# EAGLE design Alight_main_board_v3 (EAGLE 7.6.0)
CNAME: Alarm Light Main board / Juraj Repcik; CREVISION: 03
Assembly variants: ESP8266 CH340 default

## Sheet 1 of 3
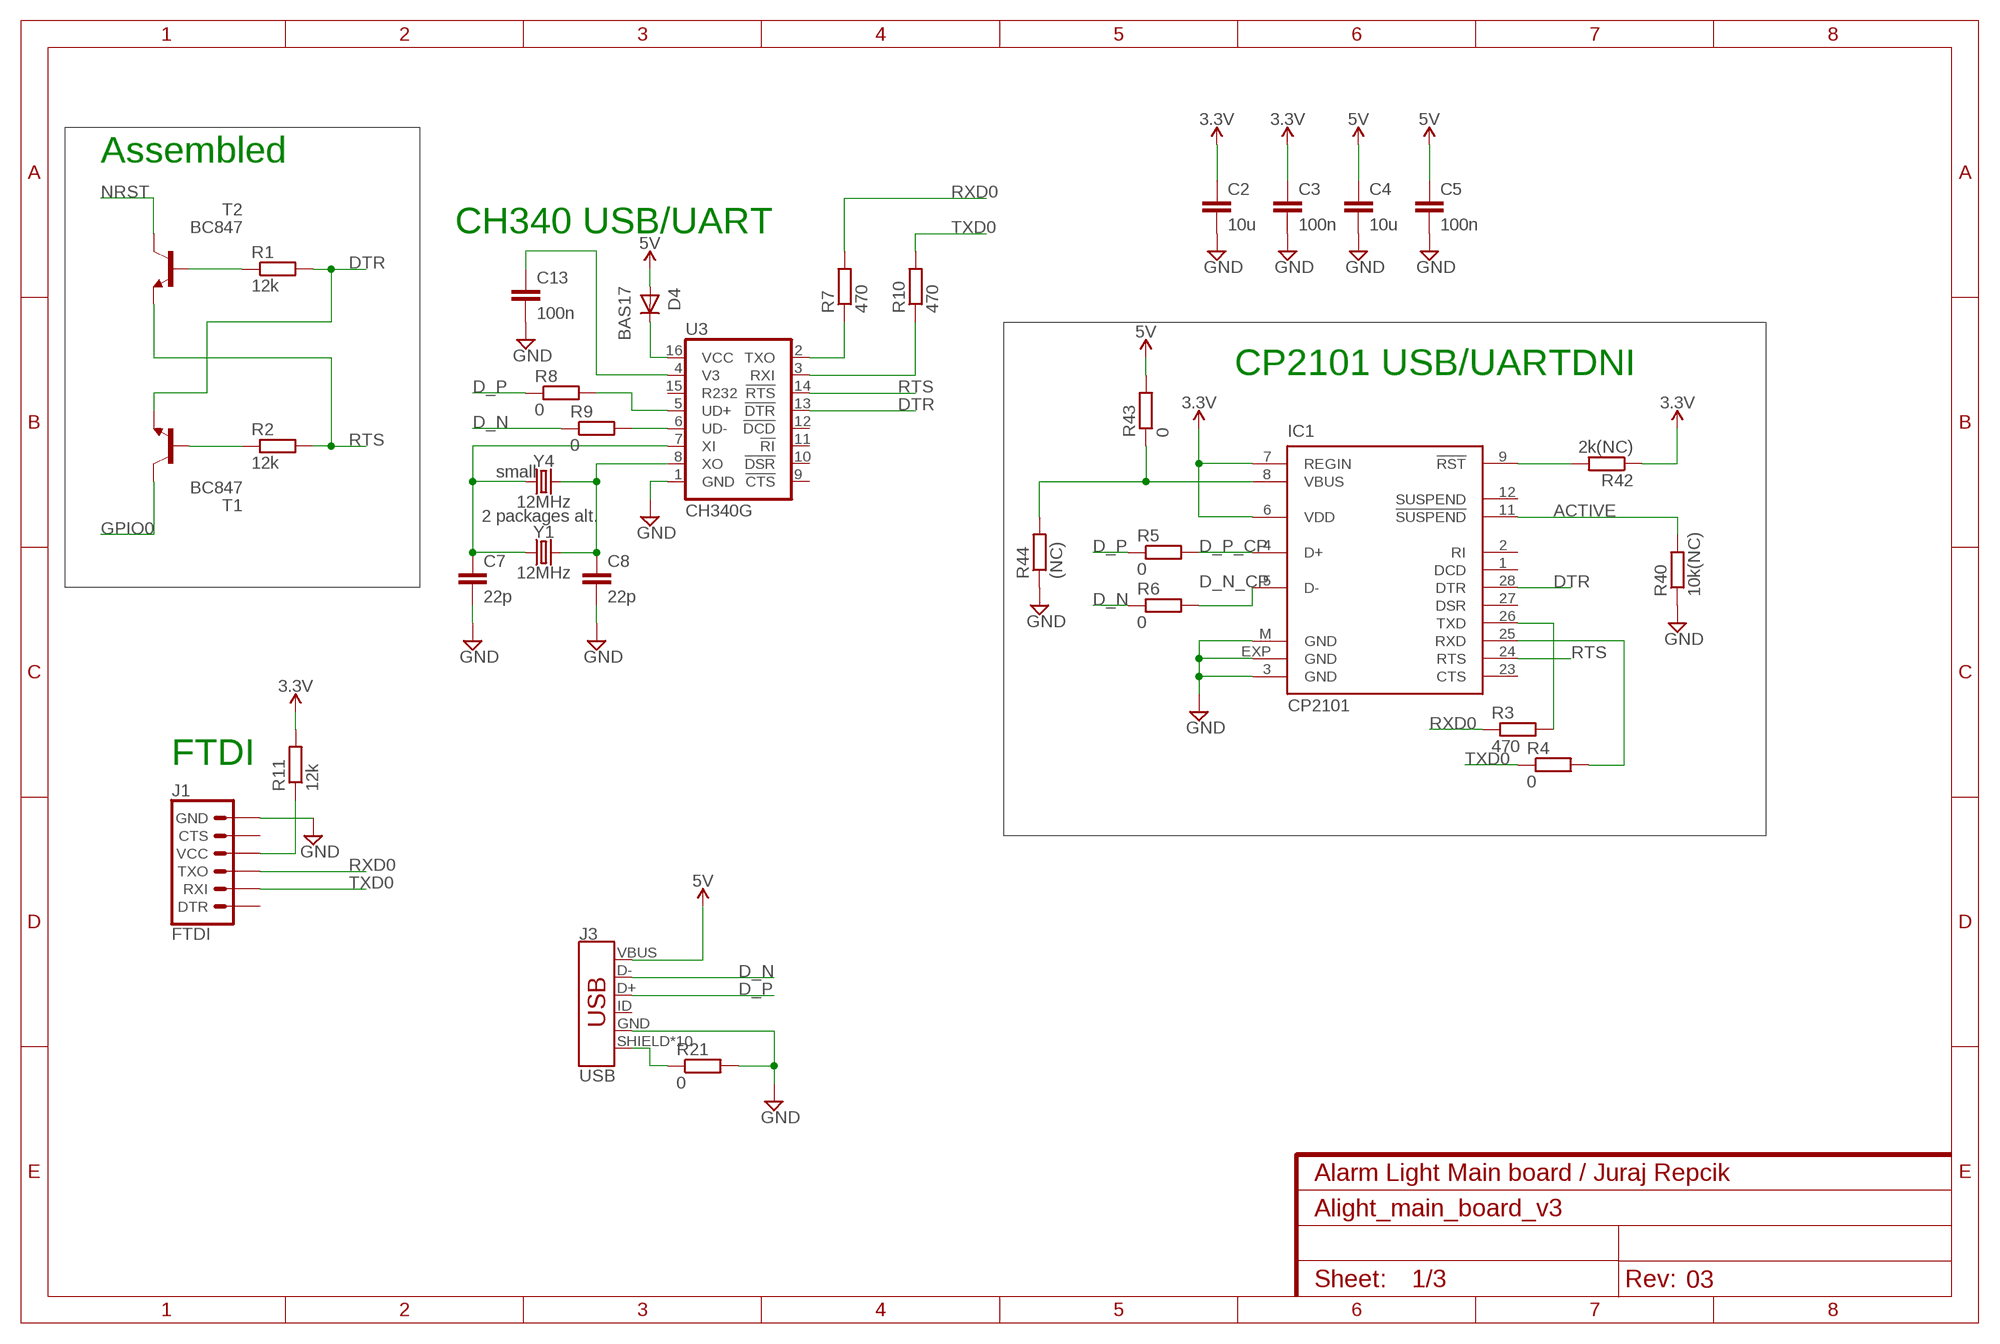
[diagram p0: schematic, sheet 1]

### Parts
C2  10u  C-EUC0603K  [C0603K]
C3  100n  C-EUC0603K  [C0603K]
C4  10u  C-EUC0603K  [C0603K]
C5  100n  C-EUC0603K  [C0603K]
C7  22p  C-EUC0402  [C0402]
C8  22p  C-EUC0402  [C0402]
C13  100n  C-EUC0603K  [C0603K]
D4  BAS17  [SOT23]
IC1  CP2101  CP210X_USB_UART  [MLP28]  (not fitted in variant ESP8266 CH340 default)
J1  FTDI  6_PIN_SERIAL_TARGETLONGPADS  [1X06_LONGPADS]
J3  USB  USB_MICRO-B_HALF_PTH_MILL  [USB-MICROB-PTH-MILL]
R1  12k  R-EU_R0603  [R0603]
R2  12k  R-EU_R0603  [R0603]
R3  470  R-EU_R0603  [R0603]  (not fitted in variant ESP8266 CH340 default)
R4  0  R-EU_R0603  [R0603]  (not fitted in variant ESP8266 CH340 default)
R5  0  R-EU_R0603  [R0603]  (not fitted in variant ESP8266 CH340 default)
R6  0  R-EU_R0603  [R0603]  (not fitted in variant ESP8266 CH340 default)
R7  470  R-EU_R0603  [R0603]
R8  0  R-EU_R0603  [R0603]
R9  0  R-EU_R0603  [R0603]
R10  470  R-EU_R0603  [R0603]
R11  12k  R-EU_R0603  [R0603]
R21  0  R-EU_R0603  [R0603]
R40  10k(NC)  R-EU_R0603  [R0603]  (not fitted in variant ESP8266 CH340 default)
R42  2k(NC)  R-EU_R0603  [R0603]  (not fitted in variant ESP8266 CH340 default)
R43  0  R-EU_R0603  [R0603]  (not fitted in variant ESP8266 CH340 default)
R44  (NC)  R-EU_R0603  [R0603]  (not fitted in variant ESP8266 CH340 default)
T1  BC847  [SOT23]
T2  BC847  [SOT23]
U3  CH340G  CH340GSMD  [SO016]
Y1  12MHz  CRYSTALSMD-HC49UP  [HC49UP]
Y4  12MHz  CRYSTAL-32.768KHZSMD-3.2X1.5  [CRYSTAL-SMD-3.2X1.5MM]  (not fitted in variant ESP8266 CH340 default)

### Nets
3.3V: C2.1 C3.1 IC1.6(VDD) IC1.7(REGIN) R11.2 R42.1 ; also sheet 2,3
5V: C4.1 C5.1 D4.1(A) J3.VBUS R43.2 ; also sheet 2,3
ACTIVE: IC1.11(!SUSPEND) R40.2
D_N: J3.D- R6.1 R9.1
D_N_CP: IC1.5(D-) R6.2
D_P: J3.D+ R5.1 R8.1
D_P_CP: IC1.4(D+) R5.2
DTR: IC1.28(DTR) R1.2 T1.2(E) U3.13(!DTR)
GND: C2.2 C3.2 C4.2 C5.2 C7.2 C8.2 C13.2 IC1.3(GND) IC1.EXP(GND) IC1.M(GND) J1.6(GND) J3.GND R21.2 R40.1 R44.1 U3.1(GND) ; also sheet 2,3
GPIO0: T1.3(C) ; also sheet 2
N$1: R1.1 T2.1(B)
N$2: R2.1 T1.1(B)
N$4: R7.1 U3.2(TXO)
N$5: R10.1 U3.3(RXI)
N$6: R8.2 U3.5(UD+)
N$7: R9.2 U3.6(UD-)
N$8: C7.1 U3.7(XI) Y1.1 Y4.P$1
N$9: C13.1 U3.4(V3)
N$10: C8.1 U3.8(XO) Y1.2 Y4.P$2
N$11: J1.4(VCC) R11.1
N$15: D4.3(K) U3.16(VCC)
N$38: IC1.9(!RST) R42.2
N$39: IC1.8(VBUS) R43.1 R44.2
NRST: T2.3(C) ; also sheet 2,3
RTS: IC1.24(RTS) R2.2 T2.2(E) U3.14(!RTS)
RXD0: J1.3(TXO) R3.1 R7.2 ; also sheet 2,3
RXD0_CP2101IN: IC1.26(TXD) R3.2
SHIELD: J3.SHIELD J3.SHIELD2(SHIELD) J3.SHIELD3(SHIELD) J3.SHIELD4(SHIELD) J3.SHIELD5(SHIELD) J3.SHIELD6(SHIELD) J3.SHIELD7(SHIELD) J3.SHIELD8(SHIELD) J3.SHIELD9(SHIELD) J3.SHIELD10(SHIELD) R21.1
TXD0: J1.2(RXI) R4.1 R10.2 ; also sheet 2,3
TXD0_CP2101: IC1.25(RXD) R4.2
Unconnected: IC1.1(DCD) IC1.2(RI) IC1.12(SUSPEND) IC1.23(CTS) IC1.27(DSR) J1.1(DTR) J1.5(CTS) J3.ID U3.9(!CTS) U3.10(!DSR) U3.11(!RI) U3.12(!DCD) U3.15(R232)

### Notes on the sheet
- Assembled
- CH340 USB/UART
- CP2101 USB/UART | DNI
- small
- 2 packages alt.
- FTDI

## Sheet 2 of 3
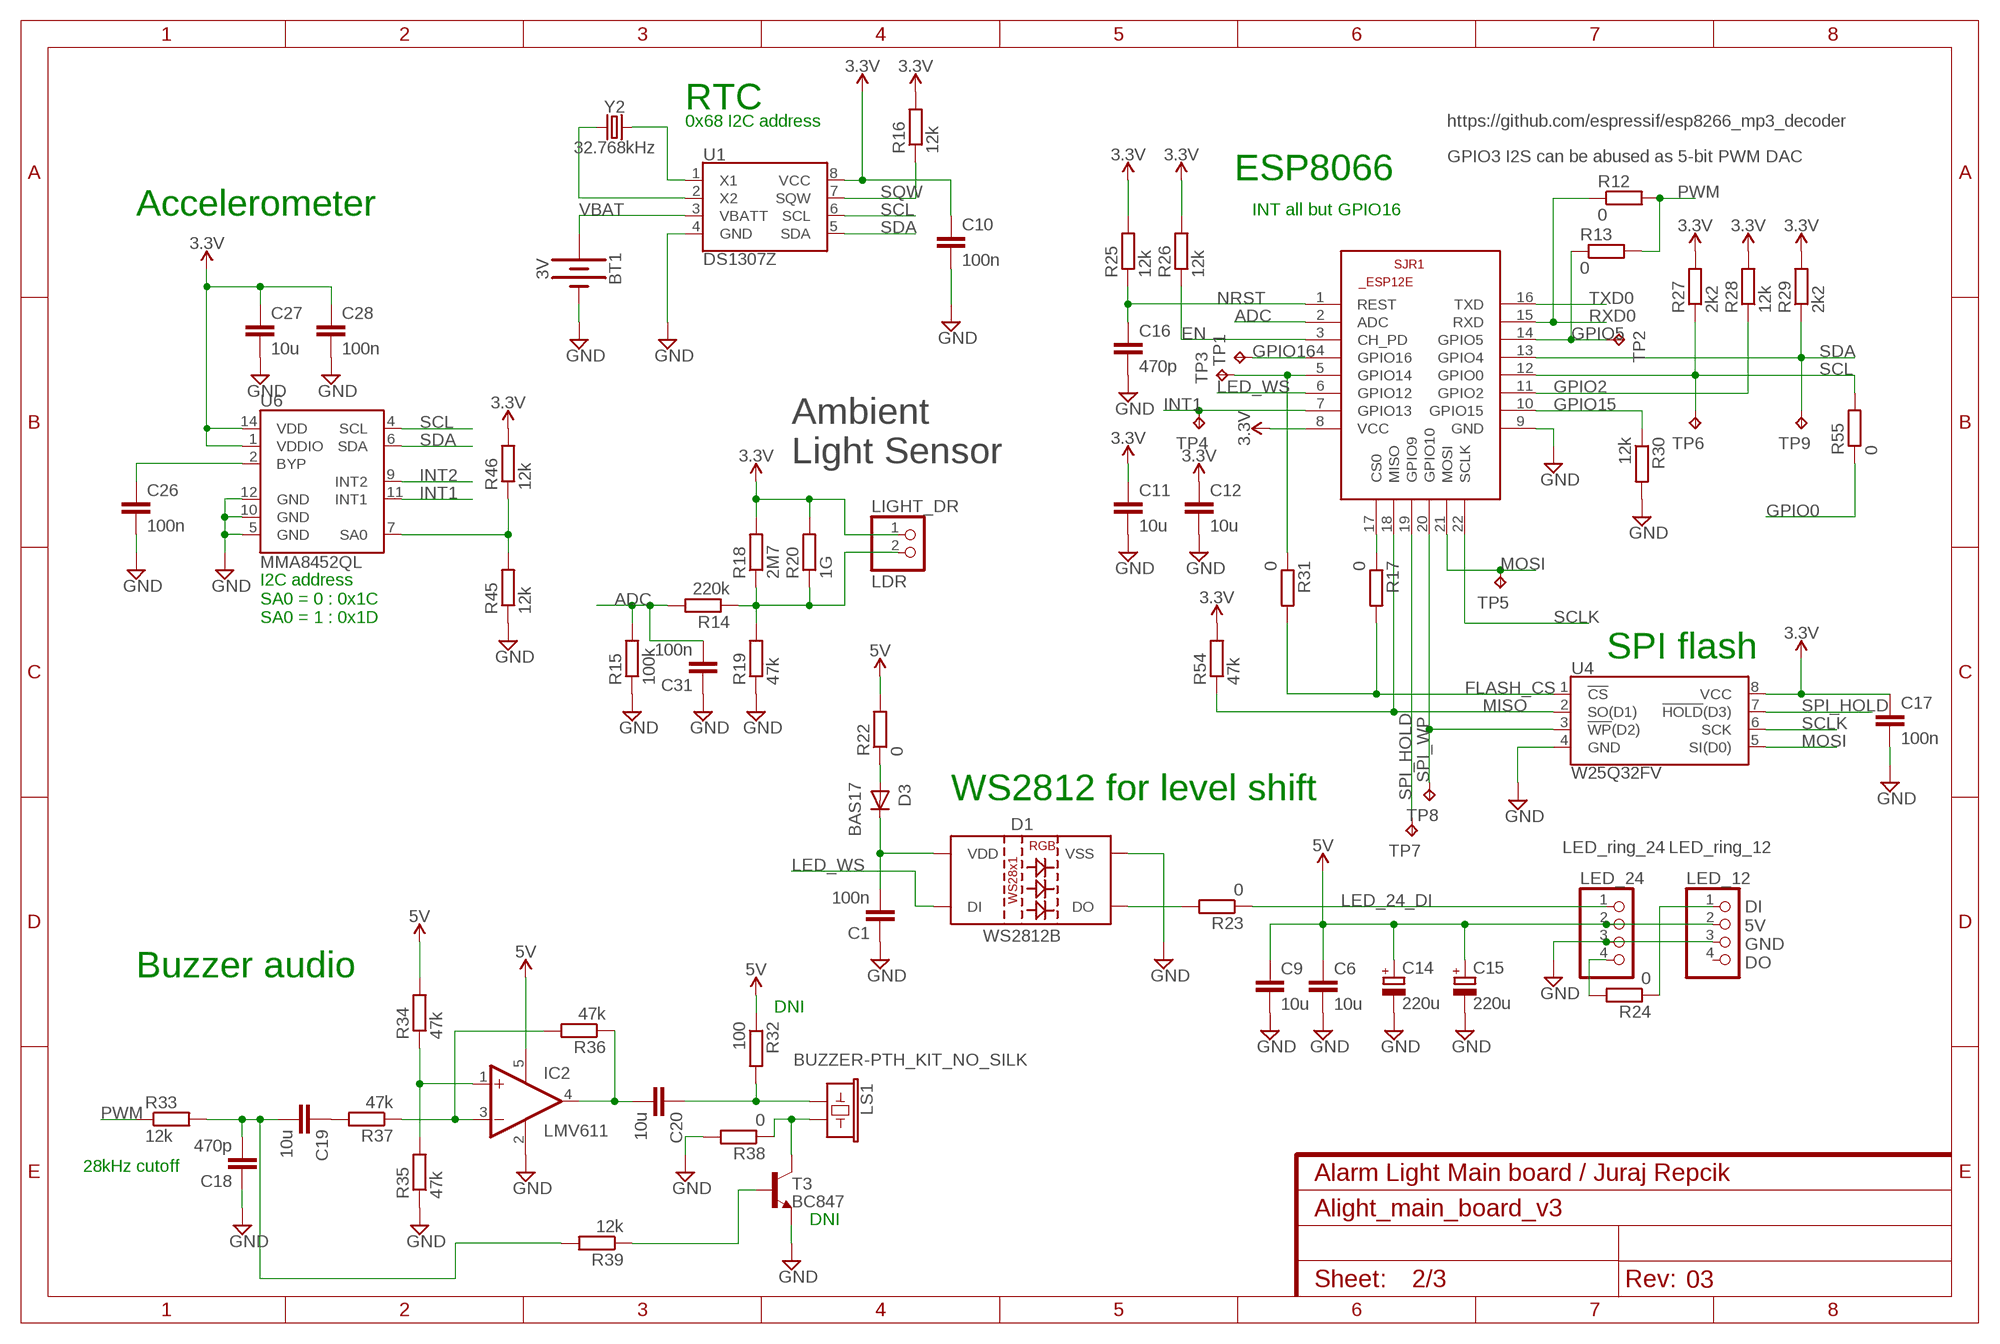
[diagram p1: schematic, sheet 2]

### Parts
BT1  3V  BATTERY-20MM_PTH_KIT  [BATTCOM_20MM_PTH_KIT]
C1  100n  C-EUC0603K  [C0603K]
C6  10u  C-EUC0603K  [C0603K]
C9  10u  C-EUC0603K  [C0603K]
C10  100n  C-EUC0603K  [C0603K]
C11  10u  C-EUC0603K  [C0603K]
C12  10u  C-EUC0603K  [C0603K]
C14  220u  CPOL-EU153CLV-0605  [153CLV-0605]
C15  220u  CPOL-EU153CLV-0605  [153CLV-0605]
C16  470p  C-EUC0603K  [C0603K]
C17  100n  C-EUC0603K  [C0603K]  (not fitted in variant ESP8266 CH340 default)
C18  470p  C-EUC0603K  [C0603K]
C19  10u  C-EUC0603K  [C0603K]
C20  10u  C-EUC0603K  [C0603K]
C26  100n  C-EUC0603K  [C0603K]
C27  10u  C-EUC0603K  [C0603K]
C28  100n  C-EUC0603K  [C0603K]
C31  100n  C-EUC0603K  [C0603K]
D1  WS2812B  [WS2812B]
D3  BAS17  [SOT23]
IC2  LMV611  OPA333DCK  [SC70-5L]
LED_12  LED_ring_12  PINHD-1X4  [1X04]
LED_24  LED_ring_24  PINHD-1X4  [1X04]
LIGHT_DR  LDR  PINHD-1X2  [1X02]
LS1  BUZZER-PTH_KIT_NO_SILK  [BUZZER-12MM-NS-KIT]
R12  0  R-EU_R0603  [R0603]  (not fitted in variant ESP8266 CH340 default)
R13  0  R-EU_R0603  [R0603]
R14  220k  R-EU_R0603  [R0603]
R15  100k  R-EU_R0603  [R0603]
R16  12k  R-EU_R0603  [R0603]
R17  0  R-EU_R0603  [R0603]  (not fitted in variant ESP8266 CH340 default)
R18  2M7  R-EU_R0603  [R0603]
R19  47k  R-EU_R0603  [R0603]
R20  1G  R-EU_R0603  [R0603]  (not fitted in variant ESP8266 CH340 default)
R22  0  R-EU_R0603  [R0603]
R23  0  R-EU_R0603  [R0603]
R24  0  R-EU_R0603  [R0603]
R25  12k  R-EU_R0603  [R0603]
R26  12k  R-EU_R0603  [R0603]
R27  2k2  R-EU_R0603  [R0603]
R28  12k  R-EU_R0603  [R0603]
R29  2k2  R-EU_R0603  [R0603]
R30  12k  R-EU_R0603  [R0603]
R31  0  R-EU_R0603  [R0603]  (not fitted in variant ESP8266 CH340 default)
R32  100  R-EU_R0603  [R0603]  (not fitted in variant ESP8266 CH340 default)
R33  12k  R-EU_R0603  [R0603]
R34  47k  R-EU_R0603  [R0603]
R35  47k  R-EU_R0603  [R0603]
R36  47k  R-EU_R0603  [R0603]
R37  47k  R-EU_R0603  [R0603]
R38  0  R-EU_R0603  [R0603]
R39  12k  R-EU_R0603  [R0603]  (not fitted in variant ESP8266 CH340 default)
R45  12k  R-EU_R0603  [R0603]  (not fitted in variant ESP8266 CH340 default)
R46  12k  R-EU_R0603  [R0603]
R54  47k  R-EU_R0603  [R0603]  (not fitted in variant ESP8266 CH340 default)
R55  0  R-EU_R0603  [R0603]
SJR1  ESP12E/F  ESP8266-12EESP12E  [ESP8266-ESP12E]
T3  BC847  [SOT23]  (not fitted in variant ESP8266 CH340 default)
TP1  TPTP10R  [TP10R]
TP2  TPTP10R  [TP10R]
TP3  TPTP10R  [TP10R]
TP4  TPTP10R  [TP10R]
TP5  TPTP10R  [TP10R]
TP6  TPTP10R  [TP10R]
TP7  TPTP10R  [TP10R]
TP8  TPTP10R  [TP10R]
TP9  TPTP10R  [TP10R]
U1  DS1307Z  [SO08-0.15]
U4  W25Q32FV  W25Q32FVSS  [SOIC-8]  (not fitted in variant ESP8266 CH340 default)
U6  MMA8452QL  [QFN-16_0.5MM-EXTRA]
Y2  32.768kHz  CRYSTAL-32.768KHZSMD-3.2X1.5  [CRYSTAL-SMD-3.2X1.5MM]

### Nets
3.3V: C10.1 C11.1 C12.1 C17.1 C27.1 C28.1 LIGHT_DR.1 R16.2 R18.2 R20.2 R25.2 R26.2 R27.2 R28.2 R29.2 R46.2 R54.2 SJR1.8(VCC) U1.8(VCC) U4.8(VCC) U6.1(VDDIO) U6.14(VDD) ; also sheet 1,3
5V: C6.1 C9.1 C14.+ C15.+ IC2.5(V+) LED_12.2 LED_24.2 R22.2 R32.1 R34.2 ; also sheet 1,3
ADC: C31.2 R14.2 R15.2 SJR1.2(ADC) ; also sheet 3
EN: R26.1 SJR1.3(CH_PD)
FLASH_CS: R17.2 R31.2 U4.1(!CS!) ; also sheet 3
GND: BT1.2(-) C1.1 C6.2 C9.2 C10.2 C11.2 C12.2 C14.- C15.- C16.2 C17.2 C18.1 C26.2 C27.2 C28.2 C31.1 D1.3(VSS) IC2.2(V-) LED_12.3 LED_24.3 R15.1 R19.1 R30.2 R35.1 R38.2 R45.1 SJR1.9(GND) T3.2(E) U1.4(GND) U4.4(GND) U6.5(GND) U6.10(GND) U6.12(GND) ; also sheet 1,3
GPIO0: R55.1 ; also sheet 1
GPIO2: R28.1 SJR1.11(GPIO2) ; also sheet 3
GPIO5: R13.1 SJR1.14(GPIO5) TP2.TP
GPIO15: R30.1 SJR1.10(GPIO15)
GPIO16: SJR1.4(GPIO16) TP1.TP
INT1: SJR1.7(GPIO13) TP4.TP U6.11(INT1) ; also sheet 3
INT2: U6.9(INT2) ; also sheet 3
LED_12DI: LED_12.1 R24.1
LED_24_DI: LED_24.1 R23.1
LED_24_DO: LED_24.4 R24.2
LED_WS: D1.4(DI) SJR1.6(GPIO12) ; also sheet 3
MISO: R54.1 SJR1.18(MISO) U4.2(SO(D1))
MOSI: SJR1.21(MOSI) TP5.TP U4.5(SI(D0))
N$3: C1.2 D1.1(VDD) D3.3(K)
N$14: LIGHT_DR.2 R14.1 R18.1 R19.2 R20.1
N$16: D3.1(A) R22.1
N$18: D1.2(DO) R23.2
N$19: C26.1 U6.2(BYP)
N$21: R31.1 SJR1.5(GPIO14) TP3.TP
N$22: R17.1 SJR1.17(CS0)
N$25: LS1.- R38.1 T3.3(C)
N$26: R39.1 T3.1(B)
N$28: IC2.1(+IN) R34.1 R35.2
N$30: U1.1(X1) Y2.P$2
N$31: U1.2(X2) Y2.P$1
N$32: IC2.3(-IN) R36.2 R37.1
N$33: C20.1 LS1.+ R32.2
N$34: C19.1 R37.2
N$35: C20.2 IC2.4(OUT) R36.1
N$36: C18.2 C19.2 R33.2 R39.2
N$40: R45.2 R46.1 U6.7(SA0)
NRST: C16.1 R25.1 SJR1.1(REST) ; also sheet 1,3
PWM: R12.2 R13.2 R33.1 ; also sheet 3
RXD0: R12.1 SJR1.15(RXD) ; also sheet 1,3
SCL: R27.1 R55.2 SJR1.12(GPIO0) TP6.TP U1.6(SCL) U6.4(SCL) ; also sheet 3
SCLK: SJR1.22(SCLK) U4.6(SCK)
SDA: R29.1 SJR1.13(GPIO4) TP9.TP U1.5(SDA) U6.6(SDA) ; also sheet 3
SPI_HOLD: SJR1.19(GPIO9) TP7.TP U4.7(!HOLD!(D3))
SPI_WP: SJR1.20(GPIO10) TP8.TP U4.3(!WP!(D2))
SQW: R16.1 U1.7(SQW)
TXD0: SJR1.16(TXD) ; also sheet 1,3
VBAT: BT1.1(+) U1.3(VBATT)
Unconnected: LED_12.4

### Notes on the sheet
- RTC
- 0x68 I2C address | https://github.com/espressif/esp8266_mp3_decoder
- GPIO3 I2S can be abused as 5-bit PWM DAC
- ESP8066
- Accelerometer | INT all but GPIO16
- Ambient
  Light Sensor
- I2C address
  SA0 = 0 : 0x1C
  SA0 = 1 : 0x1D
- SPI flash
- WS2812 for level shift
- DI
  5V
  GND
  DO
- Buzzer audio
- DNI
- 28kHz cutoff
- DNI

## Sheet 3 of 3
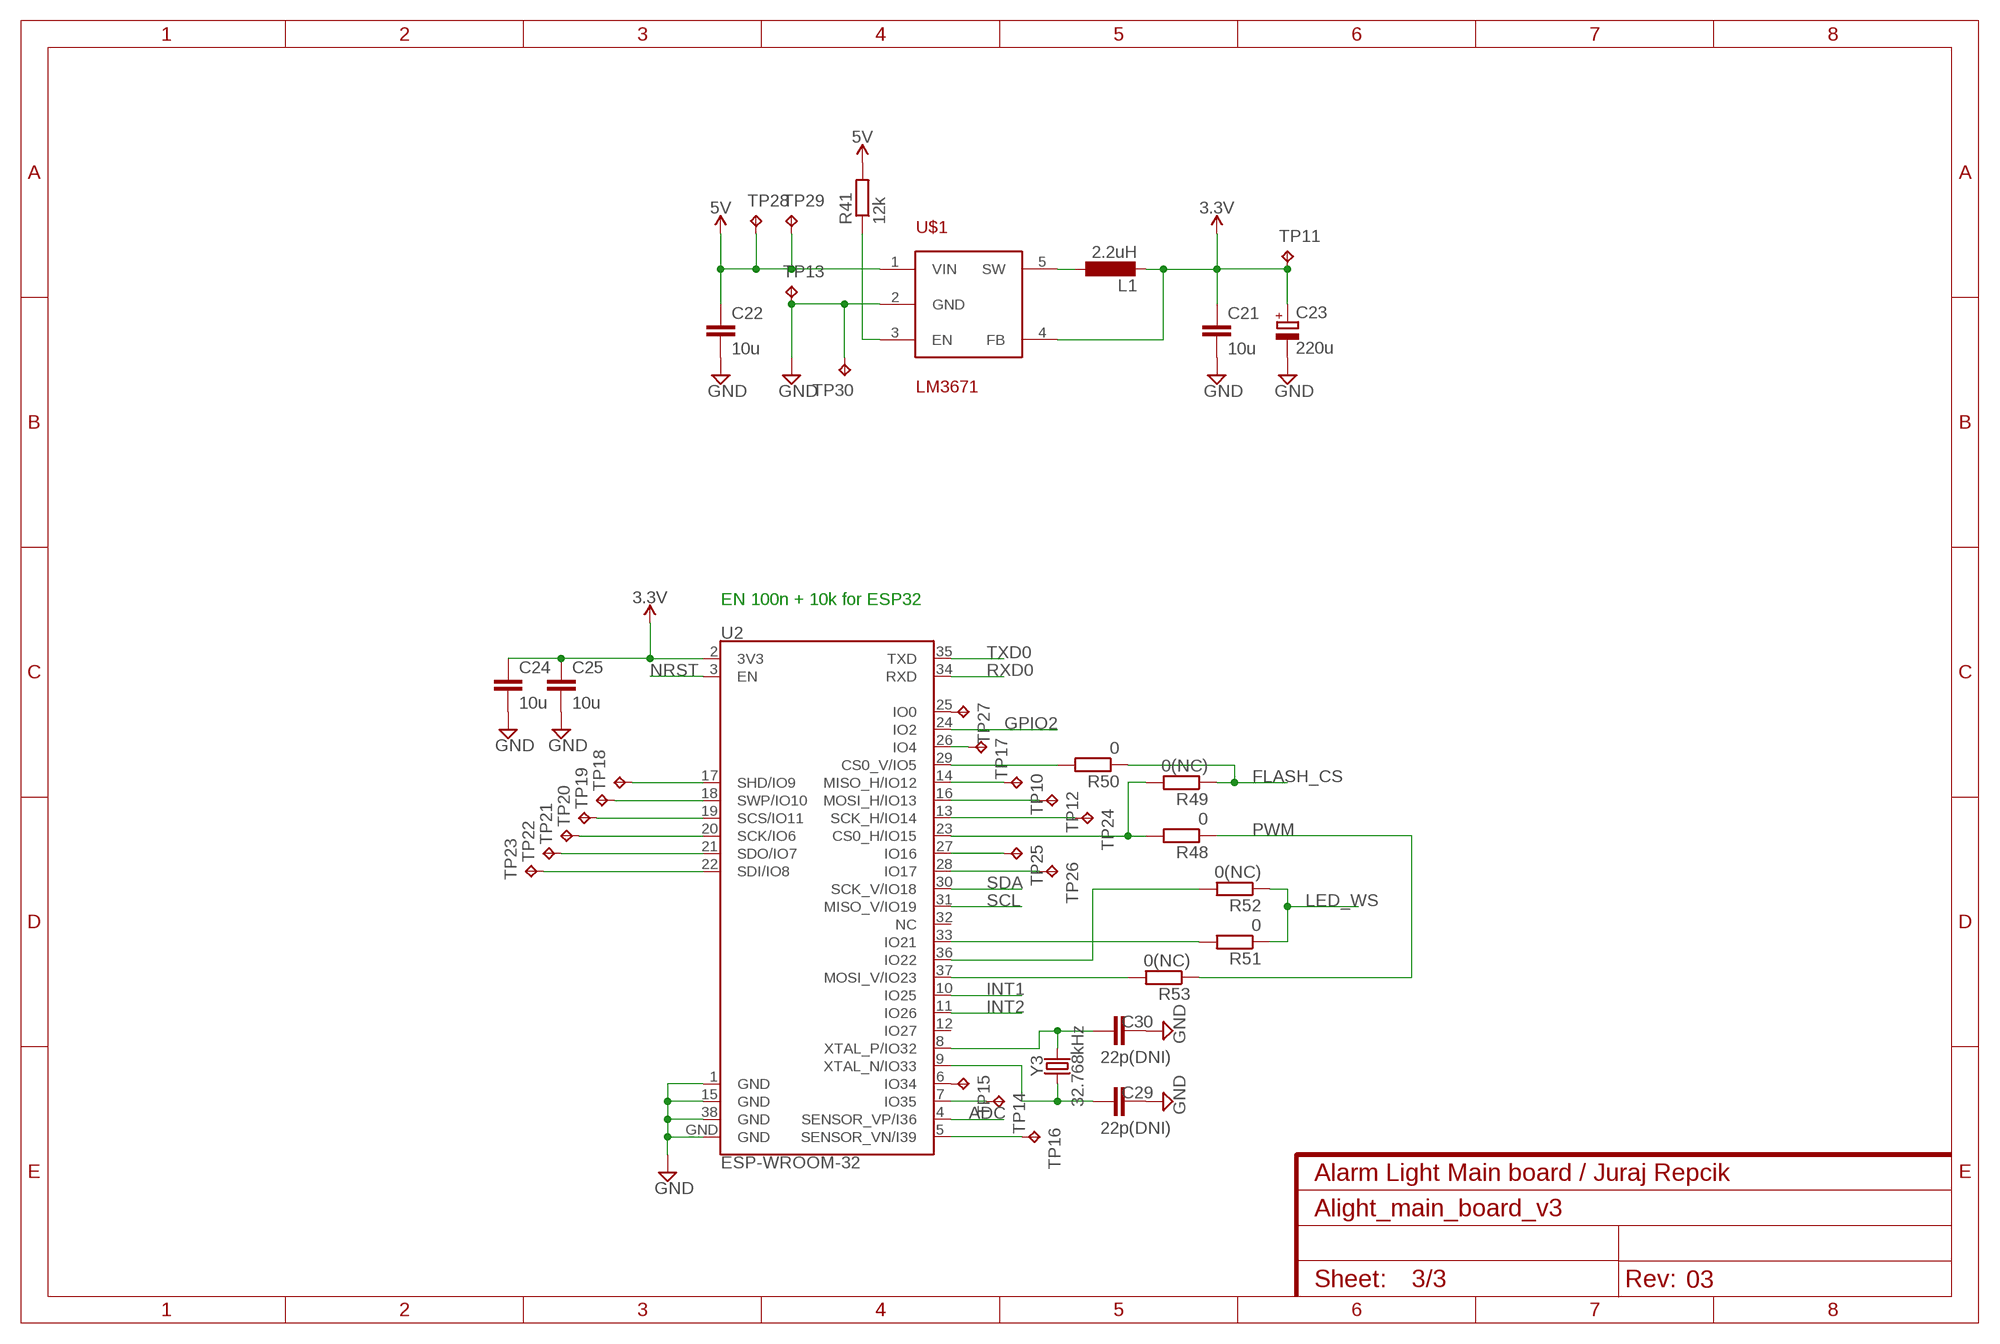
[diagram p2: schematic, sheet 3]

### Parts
C21  10u  C-EUC0603K  [C0603K]
C22  10u  C-EUC0603K  [C0603K]
C23  220u  CPOL-EU153CLV-0605  [153CLV-0605]
C24  10u  C-EUC0603K  [C0603K]  (not fitted in variant ESP8266 CH340 default)
C25  10u  C-EUC0603K  [C0603K]  (not fitted in variant ESP8266 CH340 default)
C29  22p(DNI)  C-EUC0402  [C0402]  (not fitted in variant ESP8266 CH340 default)
C30  22p(DNI)  C-EUC0402  [C0402]  (not fitted in variant ESP8266 CH340 default)
L1  2.2uH  L-EUL3225M  [L3225M]
R41  12k  R-EU_R0603  [R0603]
R48  0  R-EU_R0603  [R0603]  (not fitted in variant ESP8266 CH340 default)
R49  0(NC)  R-EU_R0603  [R0603]  (not fitted in variant ESP8266 CH340 default)
R50  0  R-EU_R0603  [R0603]  (not fitted in variant ESP8266 CH340 default)
R51  0  R-EU_R0603  [R0603]  (not fitted in variant ESP8266 CH340 default)
R52  0(NC)  R-EU_R0603  [R0603]  (not fitted in variant ESP8266 CH340 default)
R53  0(NC)  R-EU_R0603  [R0603]  (not fitted in variant ESP8266 CH340 default)
TP10  TPTP10R  [TP10R]
TP11  TPTP10R  [TP10R]
TP12  TPTP10R  [TP10R]
TP13  TPTP10R  [TP10R]
TP14  TPTP10R  [TP10R]
TP15  TPTP10R  [TP10R]
TP16  TPTP10R  [TP10R]
TP17  TPTP10R  [TP10R]
TP18  TPTP10R  [TP10R]
TP19  TPTP10R  [TP10R]
TP20  TPTP10R  [TP10R]
TP21  TPTP10R  [TP10R]
TP22  TPTP10R  [TP10R]
TP23  TPTP10R  [TP10R]
TP24  TPTP10R  [TP10R]
TP25  TPTP10R  [TP10R]
TP26  TPTP10R  [TP10R]
TP27  TPTP10R  [TP10R]
TP28  TPTP10R  [TP10R]
TP29  TPTP10R  [TP10R]
TP30  TPTP10R  [TP10R]
U2  ESP-WROOM-32  [ESP-WROOM-32]  (not fitted in variant ESP8266 CH340 default)
U$1  LM3671  [SOT23-5]
Y3  32.768kHz  CRYSTAL-32.768KHZSMD-3.2X1.5  [CRYSTAL-SMD-3.2X1.5MM]  (not fitted in variant ESP8266 CH340 default)

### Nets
3.3V: C21.1 C23.+ C24.1 C25.1 L1.2 TP11.TP U2.2(3V3) U$1.4(FB) ; also sheet 1,2
5V: C22.1 R41.2 TP28.TP TP29.TP U$1.1(VIN) ; also sheet 1,2
ADC: U2.4(SENSOR_VP/I36) ; also sheet 2
FLASH_CS: R49.1 R50.1 ; also sheet 2
GND: C21.2 C22.2 C23.- C24.2 C25.2 C29.2 C30.2 TP13.TP TP30.TP U2.1(GND) U2.15(GND) U2.38(GND) U2.GND U$1.2(GND) ; also sheet 1,2
GPIO2: U2.24(IO2) ; also sheet 2
INT1: U2.10(IO25) ; also sheet 2
INT2: U2.11(IO26) ; also sheet 2
LED_WS: R51.1 R52.1 ; also sheet 2
N$12: C30.1 U2.8(XTAL_P/IO32) Y3.P$2
N$13: C29.1 U2.9(XTAL_N/IO33) Y3.P$1
N$20: R48.2 R49.2 U2.23(CS0_H/IO15)
N$23: R51.2 U2.33(IO21)
N$24: R52.2 U2.36(IO22)
N$27: R41.1 U$1.3(EN)
N$37: L1.1 U$1.5(SW)
N$41: R50.2 U2.29(CS0_V/IO5)
N$42: R53.2 U2.37(MOSI_V/IO23)
N$43: TP14.TP U2.7(IO35)
N$44: TP15.TP U2.6(IO34)
N$45: TP16.TP U2.5(SENSOR_VN/I39)
N$46: TP17.TP U2.26(IO4)
N$47: TP18.TP U2.17(SHD/IO9)
N$48: TP19.TP U2.18(SWP/IO10)
N$49: TP20.TP U2.19(SCS/IO11)
N$50: TP21.TP U2.20(SCK/IO6)
N$51: TP22.TP U2.21(SDO/IO7)
N$52: TP23.TP U2.22(SDI/IO8)
N$63: TP10.TP U2.14(MISO_H/IO12)
N$64: TP12.TP U2.16(MOSI_H/IO13)
N$65: TP24.TP U2.13(SCK_H/IO14)
N$66: TP25.TP U2.27(IO16)
N$67: TP26.TP U2.28(IO17)
N$68: TP27.TP U2.25(IO0)
NRST: U2.3(EN) ; also sheet 1,2
PWM: R48.1 R53.1 ; also sheet 2
RXD0: U2.34(RXD) ; also sheet 1,2
SCL: U2.31(MISO_V/IO19) ; also sheet 2
SDA: U2.30(SCK_V/IO18) ; also sheet 2
TXD0: U2.35(TXD) ; also sheet 1,2
Unconnected: U2.12(IO27) U2.32(NC)

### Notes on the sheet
- EN 100n + 10k for ESP32

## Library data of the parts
BT1 = SparkFun-Batteries:BATTERY: Battery - Single Cell
C1-C13 C16-C22 C24-C31 = resistor:C-EU: CAPACITOR, European symbol
C14 C15 C23 = resistor:CPOL-EU: POLARIZED CAPACITOR, European symbol
D1 = SparkFun-LED:WS2812B: WS2812B SMD addressable RGB LED 5x5mm SMD LED with built-in controller IC. Color: Red/Green/Blue mC Rating: RGB: 390, 660, 180 mcd Forward Voltage: RGB: 2.0, 3.0, 3.0 V Packages:WS2812B SparkFun Products: Blynk Board - ESP8266; PROD_ID: DIO-12503
D3 D4 = nxp_60:BAS17: Low-voltage stabistor
IC1 = SparkFun-Retired:CP210X_USB_UART: Single-Chip USB to UART Bridge Source: www.silabs.com .. CP2101.pdf / cp2102.pdf. Spark Fun Electronics SKU : COM-00310 RETIRED: IC-00865; PROD_ID: COM-00310
IC2 = linear:OPA333: 1.8V, microPOWER CMOS OPERATIONAL AMPLIFIERS Zerø-Drift Series Source: Texas Instruments (Burr-Brown) .. U11 opa333 Operational Amp.pdf
J1 = SparkFun-Connectors:6_PIN_SERIAL_TARGET: 6-pin header connection for use with the "FTDI BASIC" pinout - TARGET SIDE. Also known as "Arduino Serial Program Header". It is used to mate with our FTDI Basic serial programmers using the Arduino IDE. Note, this device has "TARGET" in the name. It is intended to be used on a design that contains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
J3 = SparkFun-Connectors:USB_MICRO-B: USB Type Micro-B Connector Male/female and PTH/SMT variants SparkFun Products: SparkFun microB USB Breakout SparkFun USB microB Plug Breakout SparkFun ESP8266 Thing; PROD_ID: CONN-13711
L1 = resistor:L-EU: INDUCTOR, European symbol
LED_12 LED_24 = pinhead:PINHD-1X4: PIN HEADER
LIGHT_DR = pinhead:PINHD-1X2: PIN HEADER
LS1 = SparkFun-Electromechanical:BUZZER: Buzzer; PROD_ID: COMP-08253; SF_SKU: COM-07950
R1-R46 R48-R55 = resistor:R-EU_: RESISTOR, European symbol
SJR1 = esp12e:ESP8266-12E: ESP8266-12E Library for Eagle CAD The author not responsible for any damages or errors!. Created by Suhail jr.lt;/author>
T1 T2 = transistor-neu-to92:BC847: NPN TRANSISTOR
T3 = nxp_60:BC847: 45 V, 100 mA NPN general-purpose transistors NPN general-purpose transistor AAL Eindhoven MK
TP1-TP30 = testpad:TP: Test pad
U1 = SparkFun-Clocks:DS1307: Maxim DS1307 - I2C Real-time clock (RTC) The DS1307 serial real-time clock (RTC) is a low-power, full binary-coded decimal (BCD) clock/calendar plus 56 bytes of NV SRAM. Address and data are transferred serially through an I2C, bidirectional bus. The clock/calendar provides seconds, minutes, hours,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; PROD_ID: IC-08138
U2 = SparkFun-RF:ESP-WROOM-32; PROD_ID: IC-13849
U3 = SparkFun-IC-Comms:CH340G: A simple USB 2.0 to Serial IC.; PROD_ID: IC-13498
U4 = SparkFun-IC-Memory:W25Q32FV: W25Q32FV 32Mb (4MB) Serial Flash Memory The W25Q32FV support the standard Serial Peripheral Interface (SPI), Dual/Quad I/O SPI as well as 2-clocks instruction cycle Quad Peripheral Interface (QPI). 104MHz, SPI, 8-SOIC-EIAJ Datasheet SparkFun Products SparkFun Blynk Board - ESP8266 (WRL-13794); PROD_ID: IC-13229
U6 = MMA8452Q:MMA8452Q: MMA8452Q 3-Axis, 12/8-bit Digital Accelerometer Supply Voltage: 1.6-3.6V Range: +/- 2g, 4g, 8g Interface: I2C, 12-bit and 8-bit ODR: 1.56 Hz - 800 Hz Package: QFN-16 http://cache.freescale.com/files/sensors/doc/data_sheet/MMA8452Q.pdf; AVAILABILITY: Unavailable; DESCRIPTION: Sensor: accelerometer; Range: 2/4/8g; -40÷85°C; 1.95÷3.6V; MF: NXP Semiconductors; MP: MMA8452Q; PACKAGE: None; PRICE: None
U$1 = texas-custom:LM3671: Texas Instruments LM3671, LM3671Q 2MHz, 600mA Step-Down DC-DC Converter
Y1 = SparkFun-Clocks:CRYSTAL: Crystals (Generic)
Y2 Y3 = SparkFun-Clocks:CRYSTAL-32.768KHZ: 32.768kHz Crystal; PROD_ID: XTAL-13062
Y4 = SparkFun-Clocks:CRYSTAL-32.768KHZ: 32.768kHz Crystal; PROD_ID: XTAL-13062; VALUE: 32.768kHz

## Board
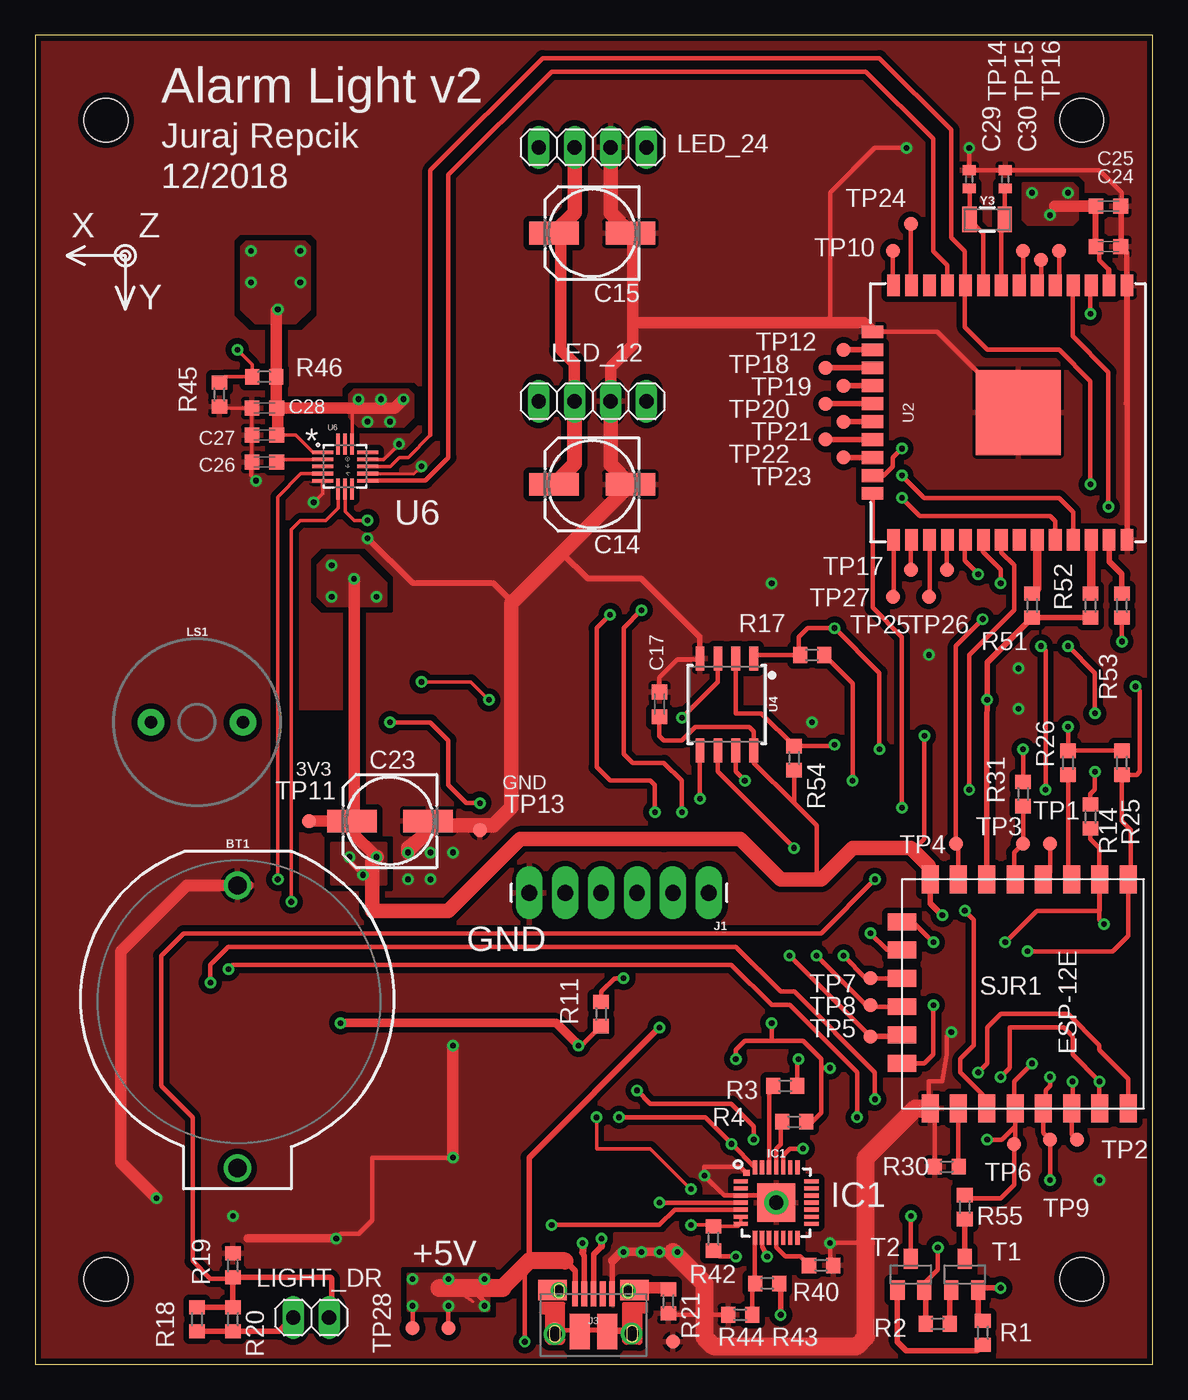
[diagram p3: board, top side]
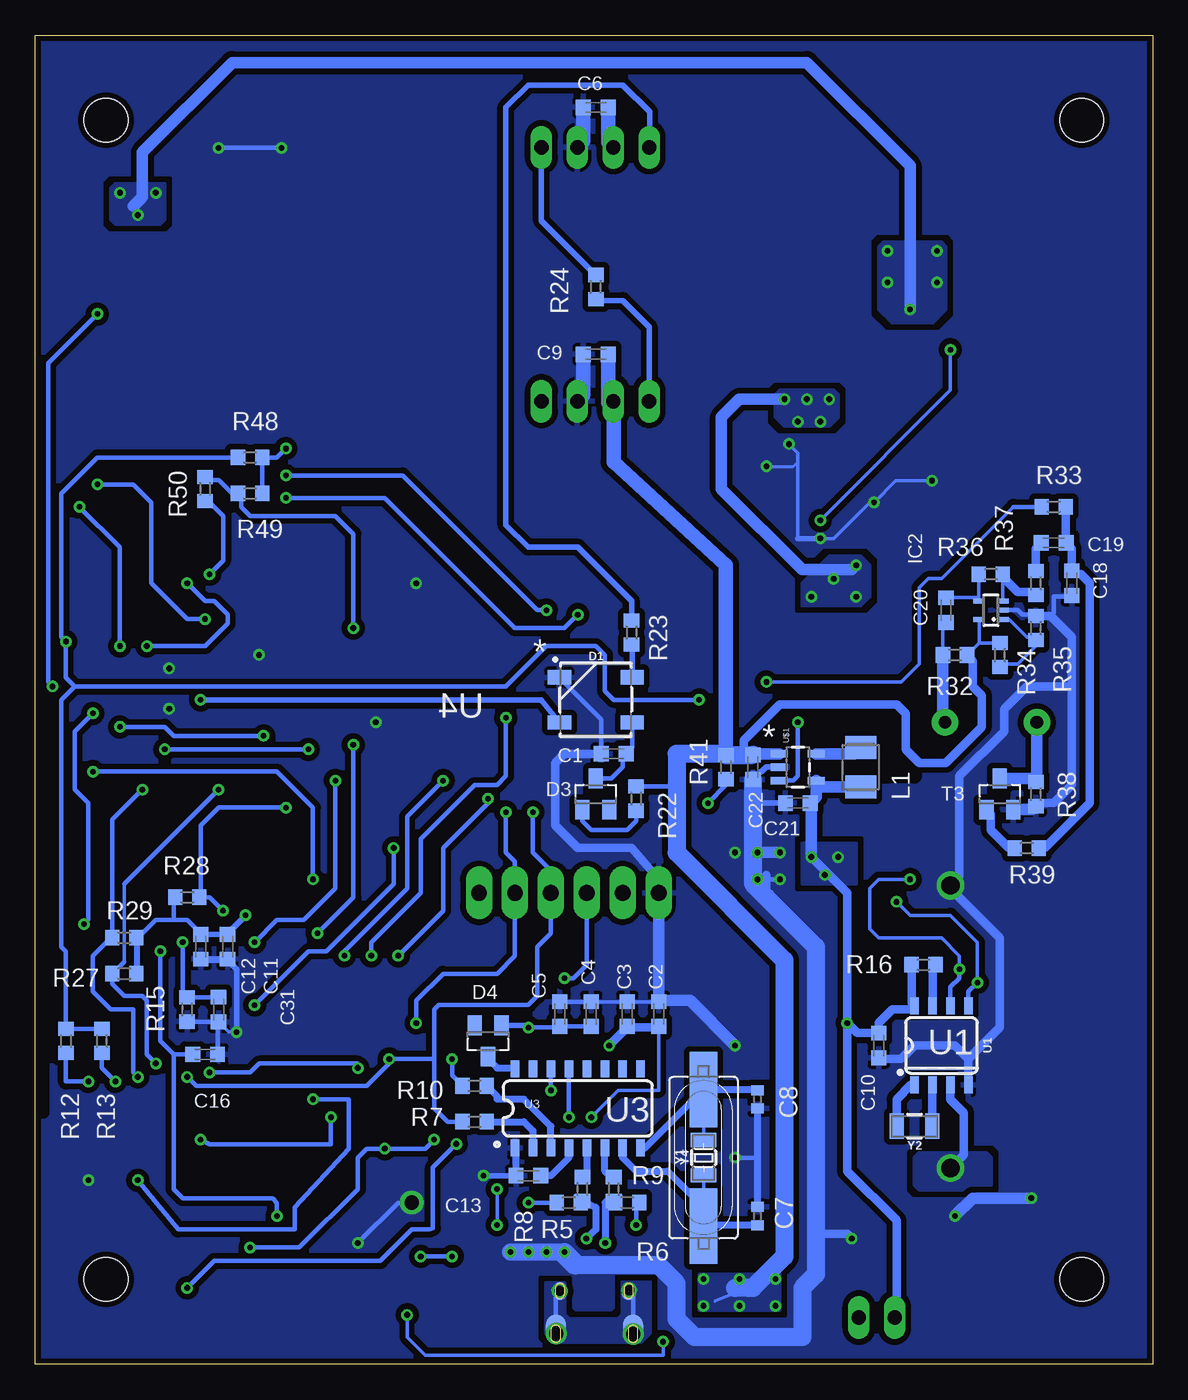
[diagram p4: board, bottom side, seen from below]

Size 79 x 94 mm. Coordinates in mm from the lower left corner, seen from the top.
Outline: 0,0 79,0 79,94 0,94 0,0
Copper layers (1*16): Top 0.035mm / dielectric 1.6mm / Bottom 0.035mm
Design rules "default *": minimum track width 8mil, minimum drill 0.399mm, track to track 6mil, track to pad 8mil, pad to pad 8mil, via to via 8mil, smd to smd 8mil, copper to edge 10mil, drill to drill 24mil, minimum pad ring 10mil, minimum via ring 8mil, stop-mask expansion 4mil, vias tented up to drill 0.59mm, thermal gap 10mil
Holes 3.1 mm at 5,6 5,88 74,88 74,6
tRestrict: area 18.7,42.2 to 21.6,45.7
bRestrict: area 16.8,41.6 to 24.1,45.7

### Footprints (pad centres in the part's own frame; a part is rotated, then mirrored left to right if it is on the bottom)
BATTCOM_20MM_PTH_KIT = drill 1.3: 1 11.85,0; 2 -8.15,0
C0603K = smd 1.05 x 1.08: 1 -0.875,0; 2 0.875,0
C0402 = smd 0.7 x 0.9: 1 -0.65,0; 2 0.65,0
153CLV-0605 = smd 3.5 x 1.6: + 2.7,0; - -2.7,0
WS2812B = smd 1.651 x 1: 1 2.577,-1.6; 2 2.577,1.6; 3 -2.577,1.6; 4 -2.577,-1.6
SOT23 = smd 1 x 1.4: 1 -0.95,-1.1; 2 0.95,-1.1; 3 0,1.1
MLP28 = smd 1 x 0.3: 1 -2.5,1.5; 2 -2.5,1; 3 -2.5,0.5; 4 -2.5,0; 5 -2.5,-0.5; 6 -2.5,-1; 7 -2.5,-1.5; 15 2.5,-1.5; 16 2.5,-1; 17 2.5,-0.5; 18 2.5,0; 19 2.5,0.5; 20 2.5,1; 21 2.5,1.5 | smd 0.3 x 1: 8 -1.5,-2.5; 9 -1,-2.5; 10 -0.5,-2.5; 11 0,-2.5; 12 0.5,-2.5; 13 1,-2.5; 14 1.5,-2.5; 22 1.5,2.5; 23 1,2.5; 24 0.5,2.5; 25 0,2.5; 26 -0.5,2.5; 27 -1,2.5; 28 -1.5,2.5 | smd 2.7 x 2.7: EXP 0,0 | smd 0.435 x 0.435: M -2.103,2.103
SC70-5L = smd 0.35 x 0.8: 1 -0.65,-0.85; 2 0,-0.85; 3 0.65,-0.85; 4 0.65,0.85; 5 -0.65,0.85
1X06_LONGPADS = drill 1.118 pad 1.88 long: 1 0,0; 2 2.54,0; 3 5.08,0; 4 7.62,0; 5 10.16,0; 6 12.7,0
USB-MICROB-PTH-MILL = smd 0.4 x 1.75: D+ 0,0; D- -0.65,0; GND 1.3,0; ID 0.65,0; VBUS -1.3,0 | smd 2 x 1.46: SHIELD -2.9,0.275; SHIELD2 2.9,0.275 | smd 1.425 x 2.5: SHIELD3 -0.963,-2.675; SHIELD4 0.963,-2.675 | smd 1.4 x 2.1 bottom: SHIELD5 -2.731,-2.531; SHIELD7 2.729,-2.531 | smd 1 x 1: SHIELD6 2.7,-2.575 | smd 1.1 x 1.5: SHIELD8 -2.731,-2.731 | smd 1 x 1.3 bottom: SHIELD9 -2.43,0.195; SHIELD10 2.43,0.195
L3225M = smd 1.6 x 2.2: 1 -1.4,0; 2 1.4,0
1X04 = drill 1.016 long: 1 -3.81,0; 2 -1.27,0; 3 1.27,0; 4 3.81,0
1X02 = drill 1.016 long: 1 -1.27,0; 2 1.27,0
BUZZER-12MM-NS-KIT = drill 0.9 pad 1.88: + 3.25,0; - -3.25,0
R0603 = smd 1 x 1.1: 1 -0.85,0; 2 0.85,0
ESP8266-ESP12E = smd 2 x 1.2: 1 -7.62,5.84; 2 -7.62,3.84; 3 -7.62,1.84; 4 -7.62,-0.16; 5 -7.62,-2.16; 6 -7.62,-4.16; 7 -7.62,-6.16; 8 -7.62,-8.16; 9 8.58,-8.16; 10 8.58,-6.16; 11 8.58,-4.16; 12 8.58,-2.16; 13 8.58,-0.16; 14 8.58,1.84; 15 8.58,3.84; 16 8.58,5.84 | smd 1.2 x 2: 17 -4.62,-10.16; 18 -2.62,-10.16; 19 -0.62,-10.16; 20 1.38,-10.16; 21 3.38,-10.16; 22 5.38,-10.16
TP10R = smd 1 x 1: TP 0,0
SO08-0.15 = smd 0.6 x 1.2: 1 -1.905,-2.8; 2 -0.635,-2.8; 3 0.635,-2.8; 4 1.905,-2.8; 5 1.905,2.8; 6 0.635,2.8; 7 -0.635,2.8; 8 -1.905,2.8
ESP-WROOM-32 = smd 0.9 x 1.5: 1 7.7,9; 2 6.43,9; 3 5.16,9; 4 3.89,9; 5 2.62,9; 6 1.35,9; 7 0.08,9; 8 -1.19,9; 9 -2.46,9; 10 -3.73,9; 11 -5,9; 12 -6.27,9; 13 -7.54,9; 14 -8.81,9; 25 -8.81,-9; 26 -7.54,-9; 27 -6.27,-9; 28 -5,-9; 29 -3.73,-9; 30 -2.46,-9; 31 -1.19,-9; 32 0.08,-9; 33 1.35,-9; 34 2.62,-9; 35 3.89,-9; 36 5.16,-9; 37 6.43,-9; 38 7.7,-9 | smd 1.5 x 0.9: 15 -10.3,5.715; 16 -10.3,4.445; 17 -10.3,3.175; 18 -10.3,1.905; 19 -10.3,0.635; 20 -10.3,-0.635; 21 -10.3,-1.905; 22 -10.3,-3.175; 23 -10.3,-4.445; 24 -10.3,-5.715 | smd 6 x 6: GND 0,0
SO016 = smd 0.6 x 1.2: 1 -4.445,-2.8; 2 -3.175,-2.8; 3 -1.905,-2.8; 4 -0.635,-2.8; 5 0.635,-2.8; 6 1.905,-2.8; 7 3.175,-2.8; 8 4.445,-2.8; 9 4.445,2.8; 10 3.175,2.8; 11 1.905,2.8; 12 0.635,2.8; 13 -0.635,2.8; 14 -1.905,2.8; 15 -3.175,2.8; 16 -4.445,2.8
SOIC-8 = smd 0.61 x 1.702: 1 -1.905,-3.251; 2 -0.635,-3.251; 3 0.635,-3.251; 4 1.905,-3.251; 5 1.905,3.251; 6 0.635,3.251; 7 -0.635,3.251; 8 -1.905,3.251
QFN-16_0.5MM-EXTRA = smd 1.5 x 0.25: 1 -1.59,1; 2 -1.59,0.5; 3 -1.59,0; 4 -1.59,-0.5; 5 -1.59,-1; 9 1.59,-1; 10 1.59,-0.5; 11 1.59,0; 12 1.59,0.5; 13 1.59,1 | smd 0.25 x 1.5: 6 -0.5,-1.59; 7 0,-1.59; 8 0.5,-1.59; 14 0.5,1.59; 15 0,1.59; 16 -0.5,1.59
SOT23-5 = smd 0.55 x 1.2: 1 -0.95,-1.3; 2 0,-1.3; 3 0.95,-1.3; 4 0.95,1.3; 5 -0.95,1.3
HC49UP = smd 5.334 x 1.93: 1 -4.826,0; 2 4.826,0
CRYSTAL-SMD-3.2X1.5MM = smd 1 x 1.8: P$1 -1.25,0; P$2 1.25,0

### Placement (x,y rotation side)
BT1  14.29,25.72 270 top
C1  38.1,43.18 0 bottom
C2  34.92,24.77 90 bottom
C3  37.15,24.77 90 bottom
C4  39.69,24.77 90 bottom
C5  41.91,24.77 90 bottom
C6  39.37,88.9 180 bottom
C7  27.94,10.48 90 bottom
C8  27.94,18.73 270 bottom
C9  39.37,71.44 180 bottom
C10  19.37,22.54 270 bottom
C11  65.41,29.53 270 bottom
C12  67.31,29.53 270 bottom
C13  44.13,13.34 180 bottom
C14  39.37,62.23 180 top
C15  39.37,80.01 180 top
C16  66.99,21.91 0 bottom
C17  44.13,46.67 90 top  (not fitted)
C18  5.71,55.24 90 bottom
C19  6.99,58.1 0 bottom
C20  14.61,53.34 90 bottom
C21  25.08,39.69 180 bottom
C22  28.26,42.23 270 bottom
C23  25.08,38.42 180 top
C24  75.88,79.06 0 top  (not fitted)
C25  75.88,81.92 0 top  (not fitted)
C26  16.19,63.82 180 top
C27  16.19,65.72 180 top
C28  16.19,67.63 180 top
C29  66.04,83.82 90 top  (not fitted)
C30  68.58,83.82 90 top  (not fitted)
C31  66.04,25.08 90 bottom
D1  39.37,46.99 0 bottom
D3  39.37,40.32 0 bottom
D4  46.99,22.86 180 bottom
DRILEGEND  [DRILEGEND]  not placed on the board
IC1  52.39,11.43 0 top  (not fitted)
IC2  11.43,53.34 90 bottom
J1  47.62,33.34 180 top
J3  39.47,4.97 0 top
L1  20.64,42.23 270 bottom
LED_12  39.4,68.11 0 top
LED_24  39.4,86.08 0 top
LIGHT_DR  19.5,3.3 0 top
LS1  11.43,45.4 0 top
R1  66.99,2.22 90 top
R2  63.82,2.86 180 top
R3  53.02,19.68 180 top  (not fitted)
R4  53.66,17.14 180 top  (not fitted)
R5  41.27,11.43 180 bottom  (not fitted)
R6  37.15,11.43 0 bottom  (not fitted)
R7  47.94,17.14 180 bottom
R8  40.32,12.38 90 bottom
R9  38.1,12.38 90 bottom
R10  47.94,19.68 180 bottom
R11  40.01,24.77 270 top
R12  76.83,22.86 90 bottom  (not fitted)
R13  74.3,22.86 90 bottom
R14  74.61,38.73 270 top
R15  68.26,25.08 90 bottom
R16  16.19,28.26 180 bottom
R17  54.93,50.16 180 top  (not fitted)
R18  11.43,3.17 270 top
R19  13.97,6.99 270 top
R20  13.97,3.17 270 top  (not fitted)
R21  44.77,4.45 270 top
R22  36.51,40.01 90 bottom
R23  36.83,51.75 270 bottom
R24  39.37,76.2 90 bottom
R25  76.83,42.55 90 top
R26  73.03,42.55 90 top
R27  72.71,27.62 0 bottom
R28  68.26,33.02 180 bottom
R29  72.71,30.16 0 bottom
R30  64.45,13.97 180 top
R31  69.85,40.32 90 top  (not fitted)
R32  13.97,50.16 180 bottom  (not fitted)
R33  6.99,60.64 0 bottom
R34  10.79,50.16 90 bottom
R35  8.26,52.07 270 bottom
R36  11.43,55.88 0 bottom
R37  8.26,55.24 90 bottom
R38  8.26,40.32 270 bottom
R39  8.89,36.51 0 bottom  (not fitted)
R40  55.56,6.99 180 top  (not fitted)
R41  30.16,42.23 90 bottom
R42  47.94,8.89 270 top  (not fitted)
R43  51.75,5.71 0 top  (not fitted)
R44  49.85,3.49 0 top  (not fitted)
R45  13.02,68.58 90 top  (not fitted)
R46  16.19,69.85 0 top
R48  63.82,64.14 0 bottom  (not fitted)
R49  63.82,61.59 0 bottom  (not fitted)
R50  66.99,61.91 270 bottom  (not fitted)
R51  70.48,53.66 90 top  (not fitted)
R52  74.61,53.66 90 top  (not fitted)
R53  76.83,53.66 90 top  (not fitted)
R54  53.66,42.86 270 top  (not fitted)
R55  65.72,11.11 90 top
SJR1  71.44,26.67 270 top
T1  65.72,6.35 0 top
T2  61.91,6.35 0 top
T3  10.79,40.32 0 bottom  (not fitted)
TP1  71.75,36.83 0 top
TP2  73.66,15.88 0 top
TP3  69.85,36.83 0 top
TP4  65.09,36.83 0 top
TP5  59.05,23.18 0 top
TP6  69.22,15.56 0 top
TP7  59.05,27.3 0 top
TP8  59.05,25.4 0 top
TP9  71.75,15.88 0 top
TP10  60.64,78.74 0 top
TP11  19.37,38.42 0 top
TP12  57.15,71.75 0 top
TP13  31.43,37.78 0 top
TP14  69.85,78.74 0 top
TP15  71.12,78.11 0 top
TP16  72.39,78.74 0 top
TP17  61.91,56.2 0 top
TP18  55.88,70.48 0 top
TP19  57.15,69.22 0 top
TP20  55.88,67.94 0 top
TP21  57.15,66.67 0 top
TP22  55.88,65.41 0 top
TP23  57.15,64.14 0 top
TP24  61.91,80.64 0 top
TP25  63.18,54.29 0 top
TP26  64.45,56.2 0 top
TP27  60.64,54.29 0 top
TP28  26.67,2.54 0 top
TP29  29.21,2.54 0 top
TP30  45.09,1.59 0 top
U1  14.92,22.54 0 bottom
U2  69.5,67.31 0 top  (not fitted)
U3  40.64,18.1 0 bottom
U4  48.9,46.67 180 top  (not fitted)
U6  21.91,63.5 0 top
U$1  25.08,42.23 270 bottom
Y1  31.75,14.61 90 bottom
Y2  16.83,16.83 180 bottom
Y3  67.31,80.96 0 top  (not fitted)
Y4  31.75,14.61 90 bottom  (not fitted)

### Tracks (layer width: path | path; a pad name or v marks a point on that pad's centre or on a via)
3.3V  (via drill 0.4 pad 0.81)
  Top 0.254: IC1.6 IC1.7 49.7,9.74 R42.1 47.84,9.84 v46.35,9.84 | v46.35,12.38 43.5,15.24 39.69,15.24 v39.69,17.46 | C27.1 18.41,65.72 19.64,64.5 U6.1 | v24.13,35.88 24.13,36.2 21.91,38.42 | U6.14 22.41,67.49 22.54,67.63
  Top 0.305: R11.2 38.63,22.54 v38.42,22.54 | 53.66,39.69 50.8,42.55 U4.8 50.8,44.77 50.48,45.09 46.67,45.09 45.72,44.13 44.45,44.13 44.13,44.45 C17.1 | 53.66,39.69 55.24,38.1 55.24,34.61 55.56,34.29 | 44.13,37.47 44.45,37.15 | R54.2 53.66,39.69 | 75.88,77.47 75.93,77.42 U2.2 75.88,76.36 75.88,77.47 | 75.25,78.82 75.25,78.11 75.88,77.47 | 75.25,78.82 C24.1 C25.1 | v73.03,45.09 R26.2 R25.2 | v62.87,44.45 62.87,37.15 62.07,36.35 | 75.25,78.82 75.25,79.06 74.93,79.38 74.93,81.92 | v22.23,35.88 22.23,35.56 v23.18,34.61 23.81,35.24 23.81,35.56
  Top 0.406: R18.2 R20.2 17.26,2.33 LIGHT_DR.1 | v64.14,31.75 63.28,32.61 SJR1.8
  Top 0.61: v38.42,22.54 36.83,24.13 v21.59,24.13
  Top 0.813: TP11.TP 21.91,38.42 C23.+ | C23.+ 22.38,37.62 v24.13,35.88 | 74.93,81.92 72.07,81.92 | v17.14,74.61 17.04,74.51 R46.2 17.04,67.65 C28.1 17.14,67.63 | v26.04,68.26 25.4,67.63 22.54,67.63 17.14,67.63 | 17.14,67.63 17.14,65.8 C27.1 | v22.54,55.56 22.54,38.58 C23.+
  Top 1.016: v24.13,35.88 23.81,35.56 23.81,32.07 29.21,32.07 34.29,37.15 44.45,37.15 49.85,37.15 52.7,34.29 55.56,34.29 57.78,36.51 61.91,36.51 62.07,36.35 63.18,35.24 63.18,34.38 SJR1.8
  Bottom 0.254: v46.35,9.84 v46.35,12.38 | v39.69,17.46 37.78,19.37 34.92,19.37 C2.1 C3.1 | L1.2 23.62,40.83 23.81,40.64 23.81,39.37 24.13,39.05
  Bottom 0.305: 37.15,23.81 C3.1 | R29.2 R27.2 71.75,27.73 71.75,30.16 70.48,31.43 69.22,31.43 | 69.22,31.43 68.26,31.43 67.31,30.48 C12.1 | R28.2 69.22,32.92 69.22,31.43 | v73.03,45.09 69.85,45.09 69.22,44.45 v62.87,44.45
  Bottom 0.406: C12.1 C11.1 65.41,30.48 v64.14,31.75
  Bottom 0.61: R16.2 17.04,25.56 U1.8 17.09,25.08 18.41,25.08 19.37,24.13 C10.1 20.88,23.42 v21.59,24.13 | C2.1 35,23.81 37.15,23.81 v38.42,22.54 | v24.13,35.88 21.59,33.34 v21.59,24.13 | LIGHT_DR.1 18.1,3.44 18.1,10.16 21.59,13.65 v21.59,24.13
  Bottom 0.813: U$1.4 23.78,40.64 | 23.78,40.64 23.78,40.11 C21.1 24.13,39.61 24.13,39.05 v24.13,35.88 | L1.2 23.59,40.83 23.78,40.64 | v17.14,74.61 17.14,84.77 24.45,92.08 65.09,92.08 71.44,85.72 71.44,82.55 72.07,81.92 | 21.27,56.2 24.77,56.2 30.48,61.91 30.48,66.99 29.21,68.26 v26.04,68.26
  other vias: 22.86,68.26 24.45,68.26 25.08,66.67 23.5,66.67 24.13,54.29 20.95,54.29 20.95,56.52 15.24,78.74 18.73,78.74 18.73,76.52 15.24,76.52 70.48,82.87 73.03,82.87 71.75,81.28
  pour Bottom (isolate 0.305): 20.95,36.83 20.95,33.97 24.77,33.97 24.77,36.83
  pour Top (isolate 0.305): 24.77,36.83 24.77,33.97 20.95,33.97 20.95,36.83
  pour Bottom (isolate 0.305): 22.23,68.58 22.54,68.9 26.35,68.9 26.67,68.58 26.67,66.99 26.04,66.36 22.86,66.36 22.23,66.99
  pour Top (isolate 0.305): 22.54,68.9 22.23,68.58 22.23,66.99 22.86,66.36 26.04,66.36 26.67,66.99 26.67,68.58 26.35,68.9
  pour Top (isolate 0.305): 20.64,57.15 20,56.52 20,54.29 20.64,53.66 24.77,53.66 24.77,55.24 22.86,57.15
  pour Bottom (isolate 0.305): 20.64,57.15 20,56.52 20,54.29 20.64,53.66 24.77,53.66 24.77,55.24 22.86,57.15
  pour Bottom (isolate 0.305): 14.92,79.38 14.61,79.06 14.61,74.61 15.56,73.66 18.41,73.66 19.37,74.61 19.37,79.06 19.05,79.38
  pour Top (isolate 0.305): 14.92,79.38 14.61,79.06 14.61,74.61 15.56,73.66 18.41,73.66 19.37,74.61 19.37,79.06 19.05,79.38
  pour Top (isolate 0.305): 69.85,83.5 69.85,80.96 70.17,80.64 73.34,80.64 73.66,80.96 73.66,83.19 73.34,83.5
  pour Bottom (isolate 0.305): 69.85,83.5 69.85,80.96 70.17,80.64 73.34,80.64 73.66,80.96 73.66,83.19 73.34,83.5 70.17,83.5
5V  (via drill 0.4 pad 0.81)
  Top 0.203: 30.94,4.45 29.53,5.4
  Top 0.305: v34.61,1.59 34.61,6.35 34.29,6.67 | 28.57,5.71 28.57,5.4 | 30.16,5.71 29.84,5.4 | 31.43,5.71 30.8,5.4 31.75,4.45 | v26.67,4.13 TP28.TP | TP29.TP v29.21,4.13
  Top 0.406: J3.VBUS 38.17,6.6 37.47,7.3 | v44.13,23.81 34.92,14.61 34.92,7.3 | R43.2 52.7,5.61 v52.7,3.49
  Top 0.813: C15.+ 37.15,79.53 37.15,71.75 38.1,70.8 38.1,67.94 38.1,67.63 38.13,67.66 LED_12.2
  Top 1.016: LED_24.2 38.13,81.47 C15.+ | LED_12.2 38.13,63.69 C14.+ 38.1,63.66 38.1,67.94
  Top 1.2: 37.47,7.3 34.92,7.3 34.29,6.67 33.02,5.4
  Top 1.27: 28.57,5.4 29.53,5.4 29.84,5.4 33.02,5.4
  Bottom 0.203: 28.57,5.4 30.94,4.45
  Bottom 0.254: R34.2 12.27,51.02 | 12.27,51.02 R32.1 | 12.27,51.02 IC2.5 | v34.61,1.59 34.61,0.64 51.44,0.64 52.7,1.91 v52.7,3.49
  Bottom 0.305: C4.1 C5.1 41.99,23.81 v44.13,23.81 | R22.2 33.76,40.85 33.66,40.96
  Bottom 0.406: D4.1 44.28,23.96 v44.13,23.81
  Bottom 0.61: R32.1 12.7,49.74 12.7,47.94 12.06,47.31 12.06,45.09 14.61,42.55 16.51,42.55 17.46,43.5 17.46,46.04 18.1,46.67 26.35,46.67 28.89,44.13 28.89,43.1
  Bottom 0.813: U$1.1 28.18,43.18 C22.1
  Bottom 1.016: C6.1 38.49,86.44 LED_24.2 | C9.1 38.49,68.02 38.1,67.63 | 38.1,67.63 38.1,68.08 LED_12.2 | 38.1,67.63 38.1,63.82 30.16,56.52 30.16,43.18
  Bottom 1.27: C22.1 28.89,43.1 30.14,43.1 R41.2 30.27,43.18 | 30.27,43.18 30.16,43.18 | 30.27,43.18 33.66,43.18 33.66,40.96 33.66,36.2 26.04,28.57 26.04,7.62 28.26,5.4 28.57,5.4 29.53,5.4
  other vias: 26.67,6.03 29.21,6.03 31.75,6.03 31.75,4.13
  pour Top (isolate 0.305): 26.35,6.35 26.35,3.81 32.07,3.81 32.07,6.35
  pour Bottom (isolate 0.305): 26.35,6.35 26.35,3.81 32.07,3.81 32.07,6.35
ACTIVE
  Top 0.305: R40.2 54.08,7.62 53.02,7.62 52.39,8.26 IC1.11
ADC  (via drill 0.4 pad 0.81)
  Top 0.305: 75.25,34.32 SJR1.2 75.28,32.1 75.25,32.07 | v68.58,29.84 70.8,32.07 75.25,32.07 | 75.25,34.32 75.25,36.51 74.61,37.15 R14.2 | 75.25,34.32 75.25,32.07 | 75.25,32.07 75.25,31.43 v75.56,31.11 | U2.4 73.34,76.26 73.34,72.71 75.88,70.17 v75.88,60.64 | v73.03,50.8 74.93,48.9 v74.93,46.04
  Bottom 0.305: C31.2 68.24,25.96 R15.2 68.58,26.25 v68.58,29.84 | v75.56,31.11 75.25,31.43 75.25,39.69 76.2,40.64 76.2,44.77 v74.93,46.04 | v73.03,50.8 73.03,57.78 v75.88,60.64
D_N  (via drill 0.4 pad 0.82)
  Top 0.406: 38.7,7.9 38.82,7.61 38.82,5.05 J3.D-
  Top 0.5: v38.7,8.57 38.7,7.9
  Bottom 0.203: R6.1 R9.1
  Bottom 0.5: R9.1 38.6,11.53 38.7,11.43 v38.7,8.57
D_N_CP  (via drill 0.4 pad 0.81)
  Top 0.305: IC1.5 45.22,10.93 44.13,9.84 v36.51,9.84
  Bottom 0.305: v36.51,9.84 36.51,11.21 R6.2
D_P  (via drill 0.4 pad 0.81)
  Top 0.406: 40.04,8.32 39.48,7.77 39.48,4.99 J3.D+
  Top 0.5: 40.04,8.32 v40.04,8.89
  Bottom 0.203: R5.1 R8.1
  Bottom 0.5: R8.1 40.14,11.53 39.4,11.11 39.37,11.08 39.37,9.53 40.01,8.89 v40.04,8.89
D_P_CP  (via drill 0.4 pad 0.81)
  Top 0.305: IC1.4 v44.13,11.43
  Bottom 0.305: v44.13,11.43 R5.2
DTR  (via drill 0.4 pad 0.81)
  Top 0.305: v41.27,17.46 47.35,17.46 v49.24,15.58 IC1.28
  Top 0.406: R1.2 66.67,3.39 T1.2 66.82,5.4 v68.26,5.4
  Bottom 0.305: v41.27,17.46 U3.13 | v68.26,5.4 66.36,7.3 54.61,7.3 52.39,9.53 51.12,9.53 50.89,9.61 IC1.28 v49.24,15.58
EN
  Top 0.305: SJR1.3 73.03,34.54 R26.1
FLASH_CS  (via drill 0.4 pad 0.81)
  Top 0.305: U4.1 51.04,50.16 R17.2 53.98,50.27 53.98,51.44 54.61,52.07 v56.52,52.07 59.69,48.9 v59.69,43.5 | R31.2 v69.85,43.5
  Bottom 0.305: v69.85,43.5 v59.69,43.5 | R50.1 66.78,62.55 66.04,62.55 65.09,61.59 R49.1 64.45,61.38 64.45,60.64 63.82,60.01 57.78,60.01 56.52,58.74 v56.52,52.07
GND  (via drill 0.4 pad 0.81, 1 pad 1.68)
  Top 0.203: U6.10 26.8,63 v27.3,63.5
  Top 0.254: 45.09,7.94 47.62,5.4 47.62,1.59 | C26.2 15.24,63.74 15.24,62.87 v15.61,62.5 15.32,62.79 C26.2 | C26.2 C27.2 C28.2 13.12,67.63 R45.1 | v25.72,65.09 24.63,64 U6.12 | TP13.TP 31.43,38.1 | U6.5 20.32,61.59 v19.68,60.96 20.32,61.59 U6.5
  Top 0.305: IC1.EXP 51.89,11.93 IC1.3 48.71,11.93 v47.31,13.34 47.31,13.97 49.85,13.97 IC1.M | R40.1 56.2,7.2 v56.2,8.57 58.74,8.57 | R44.1 47.31,3.49 44.87,3.49 R21.2 | SJR1.9 63.6,17.77 R30.2 | v29.53,14.61 23.81,14.61 23.81,10.16 22.86,9.21 21.59,9.21 v21.27,8.89 | 63.18,18.18 63.73,18.18 | C17.2 44.13,48.58 45.4,49.85 46.91,49.85 U4.4 | U2.15 63.78,73.03 U2.GND | C29.2 C30.2 75.23,84.47 75.25,84.45 | U2.1 77.2,78.61 C24.2 C25.2 76.83,81.99 | 76.83,81.99 76.83,82.87 75.25,84.45 | 77.15,67.94 77.15,79.06 76.83,79.38 76.83,81.99 | 75.25,84.45 66.04,84.45 v66.04,86.04 | v61.59,86.04 59.37,86.04 56.2,82.87 56.2,73.66 | v64.77,23.5 64.45,23.18 64.45,21.91 64.14,20 63.18,20 63.18,18.1 63.82,18.1
  Top 0.406: J3.GND 40.79,4.99 40.79,7.3 | SJR1.9 63.18,18.18 | U2.38 77.2,67.9 77.15,67.94 77.2,67.99 U2.1 | U2.GND 70.14,67.94 | 33.66,53.81 33.66,53.98 32.38,55.24 26.67,55.24 v23.5,58.42 | U4.4 46.99,51.44 42.86,55.56 39.05,55.56 37.23,57.39 | 33.97,53.02 33.66,53.34
  Top 0.61: 40.79,7.3 41.43,7.94 v41.59,7.94 v42.86,7.94 v44.13,7.94 45.09,7.94 | 15.03,8.89 v21.27,8.89 | 15.03,33.87 BT1.2
  Top 0.813: C23.- 27.78,37.62 v26.35,36.2 | C15.- 42.23,79.85 42.23,73.66 | LED_12.3 40.67,70.52 42.23,72.07 42.23,73.66 | 15.03,33.87 10.69,33.87 6.03,29.21 6.03,14.29 v8.57,11.75 | v29.53,22.54 v29.53,14.61 | 42.23,73.66 56.2,73.66 58.56,73.66 U2.15
  Top 1.016: LED_24.3 40.67,81.41 C15.- | LED_12.3 40.67,63.63 C14.- 37.23,57.39 33.66,53.81 33.66,53.34 33.66,39.37 32.38,38.1 31.43,38.1 28.26,38.1 27.78,37.62 26.35,36.51 v26.35,36.2
  Top 1.27: 45.09,7.94 47.31,5.71 47.31,3.49 47.31,1.91 47.62,1.59 47.94,1.27 58.1,1.27 58.74,1.91 58.74,8.57 58.74,14.61 62.22,18.09 SJR1.9
  Bottom 0.203: v27.3,63.5 25.4,63.5 25.08,63.82
  Bottom 0.254: C2.2 C3.2 C4.2 | C31.1 65.33,23.5 v64.77,23.5 | v15.61,62.5 18.14,62.5 v19.68,60.96 20,60.96 22.54,58.42 v23.5,58.42 | 25.08,58.42 25.08,63.82 25.08,64.45 v25.72,65.09
  Bottom 0.305: R15.1 68.24,24.21 C31.1 66.12,24.13 C16.2 | C5.2 C4.2 | v56.2,8.57 53.34,11.43 IC1.EXP | C1.1 38.98,45.62 D1.3 | 27.94,14.61 v29.53,14.61 | v66.04,86.04 v61.59,86.04 | v26.35,34.29 26.99,34.29 27.3,34.61 | R35.1 8.36,53.02 9.21,53.02 9.53,53.34 IC2.2 | 7.2,52.92 6.99,53.13 6.99,54.29 5.71,54.29
  Bottom 0.406: C13.2 v47.31,13.34 | U$1.2 27.3,42.23 27.62,41.91 27.7,41.91 C22.2 | 28.26,39.69 C21.2 | C11.2 C12.2 67.23,28.57 65.41,28.57 64.77,27.94 v64.77,23.5 | v23.5,58.42 25.08,58.42
  Bottom 0.5: C8.2 27.94,14.61 C7.2 | C13.2 45.01,15.22 U3.1
  Bottom 0.61: R35.1 7.2,52.92 5.71,51.44 5.71,47.94 | 5.71,47.94 5.71,40.96 6.99,39.69 8.04,39.69 R38.2 | C18.1 5.75,54.37 | U1.4 13.02,21.59 | 13.02,21.59 13.97,22.54 16.83,22.54 17.78,21.59 19.29,21.59 C10.2 | 13.02,21.59 10.79,23.81 10.79,30.16 14.29,33.66 BT1.2 13.65,34.5 13.65,41.59 10.48,44.77 10.48,46.35 8.89,47.94 5.71,47.94 | C1.1 41.59,43.18 42.23,42.55 42.23,38.1 40.64,36.51 36.83,36.51 34.92,34.29 J1.6 | v21.27,8.89 21.59,9.21 23.81,9.21 | 27.3,33.02 27.3,34.61
  Bottom 0.813: T3.2 8.51,39.22 R38.2 | C2.2 34.92,25.72 | v26.35,36.2 v27.94,36.2 28.26,36.2 | v8.57,11.75 12.7,11.75 v13.97,10.48 | J1.6 34.92,25.72 | 34.92,25.72 32.7,25.72 v29.53,22.54
  Bottom 1.016: C6.2 40.24,86.51 LED_24.3 | C9.2 40.24,68.54 LED_12.3
  Bottom 1.2: v45.4,7.94 41.91,7.94 40.96,6.99 34.92,6.99
  Bottom 1.27: C22.2 28.26,39.69 28.26,36.2 28.26,33.97 27.3,33.02 23.81,29.53 23.81,9.21 23.81,6.35 24.77,5.4 24.77,1.91 32.38,1.91 33.66,3.17 33.66,5.71 34.92,6.99 40.79,6.99 40.79,7.13 v41.59,7.94
  other vias: 52.39,11.43 29.53,36.2 27.94,34.29 52.07,55.24 63.18,50.16 69.53,49.21 69.53,46.35 54.93,45.4 75.25,13.02
  pour Top (isolate 0.305): 40.96,9.21 40.96,6.67 46.04,6.67 46.04,8.57 45.4,9.21
  pour Bottom (isolate 0.305): 40.96,9.21 40.96,6.67 46.04,6.67 46.04,8.57 45.4,9.21
  pour Top (isolate 0.305): 25.72,36.83 25.72,33.97 28.89,33.97 29.84,34.92 29.84,36.83
  pour Bottom (isolate 0.305): 25.72,36.83 25.72,33.97 28.89,33.97 29.84,34.92 29.84,36.83
  pour Top (isolate 0.406, rank 2): 0,94 0,0 79,0 79,94
  pour Bottom (isolate 0.406, no thermals): 15.88,33.97 15.88,33.02 15.56,32.7 12.06,32.7 11.75,33.02 11.75,34.61 12.06,34.92 15.56,34.92 15.88,34.61
  pour Bottom (isolate 0.406, rank 2): 0,94 0,0 79,0 79,94
GPIO0
  Top 0.406: R55.1 T1.3
GPIO2  (via drill 0.4 pad 0.81)
  Top 0.305: 67.31,18.06 SJR1.11 66.99,18.38 66.99,19.05 65.41,20.64 65.41,21.59 66.36,22.54 66.36,31.43 v65.72,32.07 | U2.24 59.2,53.51 61.28,51.44 v61.28,39.37
  Bottom 0.305: v65.72,32.07 66.67,33.02 R28.1 67.31,33.12 67.31,38.1 66.04,39.37 v61.28,39.37
GPIO5  (via drill 0.4 pad 0.81)
  Top 0.305: v73.34,20 73.34,18.16 SJR1.14 73.28,16.26 TP2.TP
  Bottom 0.305: v73.34,20 74.3,20.95 R13.1
GPIO15
  Top 0.305: R30.1 65.28,14.95 SJR1.10
GPIO16
  Top 0.305: TP1.TP 71.75,34.77 SJR1.4
INT1  (via drill 0.4 pad 0.81)
  Top 0.254: U6.11 25.08,63.5 25.72,64.14 26.35,64.14 27.94,65.72
  Top 0.305: SJR1.7 65.28,36.64 TP4.TP 65.09,50.8 v66.99,52.7 | v74.61,62.23 74.61,69.53 72.39,71.75 67.31,71.75 65.72,73.34 65.72,76.26 U2.10 65.72,76.36 65.72,78.74 64.77,79.69 64.77,87.31 59.69,92.39 35.88,92.39 27.94,84.45 27.94,65.72
  Bottom 0.305: v74.61,62.23 72.07,62.23 70.8,60.96 70.8,55.24 68.26,52.7 v66.99,52.7
INT2
  Top 0.305: U6.9 27.57,62.5 29.21,64.14 29.21,84.14 36.51,91.44 58.74,91.44 63.5,86.68 63.5,78.74 64.5,77.74 U2.11
LED_12DI
  Bottom 0.406: R24.1 39.27,75.25 37.47,75.25 35.59,73.38 LED_12.1
LED_24_DI
  Bottom 0.406: R23.1 36.83,53.98 40.64,57.78 44.13,57.78 45.72,59.37 45.72,88.9 44.13,90.49 37.47,90.49 35.56,88.58 35.56,86.11 LED_24.1
LED_24_DO
  Bottom 0.406: R24.2 43.21,80.89 LED_24.4
LED_WS  (via drill 0.4 pad 0.81)
  Top 0.406: SJR1.6 67.28,45.37 v67.31,46.99 67.31,49.63 R51.1 R52.1
  Bottom 0.406: v67.31,46.99 43.23,46.99 D1.4
  Bottom 0.61: D1.4 41.96,45.4
MISO  (via drill 0.4 pad 0.81)
  Top 0.305: SJR1.18 60.24,29.29 v59.05,30.48 | v56.52,43.81 56.41,43.71 R54.1 51.33,46.04 49.53,46.04 U4.2
  Bottom 0.305: v59.05,30.48 56.52,33.02 v56.52,43.81
MOSI  (via drill 0.4 pad 0.81)
  Top 0.305: TP5.TP v53.34,28.89 | v46.99,40.01 U4.5
  Top 0.406: TP5.TP 61.16,23.18 SJR1.21
  Bottom 0.305: v46.99,40.01 46.99,39.69 50.16,36.51 50.16,32.07 v53.34,28.89
N$1
  Top 0.406: R1.1 66.57,0.95 61.59,0.95 60.96,1.58 T2.1
N$2
  Top 0.406: T1.1 64.67,5.14 R2.1
N$3
  Bottom 0.305: D3.3 38.27,41.42 37.47,42.23 37.47,42.94 C1.2 36.79,43.61 D1.1
N$4
  Bottom 0.5: R7.1 44.45,17.14 43.81,16.51 U3.2
N$5
  Bottom 0.5: U3.3 42.55,16.83 44.45,18.73 46.35,18.73 46.35,18.95 R10.1
N$6
  Bottom 0.5: U3.5 40.01,13.55 R8.2
N$7
  Bottom 0.5: R9.2 38.31,13.23 38.73,13.65 U3.6
N$8
  Bottom 0.254: Y4.P$1 31.75,12.06 32.23,11.59
  Bottom 0.5: U3.7 37.47,14.61 36.51,13.65 34.29,13.65 32.23,11.59 31.75,11.11 Y1.1 31.7,9.83 C7.1
N$9
  Bottom 0.5: U3.4 41.27,14.61 42.55,13.34 C13.1
N$10
  Bottom 0.254: Y4.P$2 31.75,18.41 32.1,18.76 32.42,18.76
  Bottom 0.5: U3.8 35.88,15.3 32.42,18.76 Y1.2 27.99,19.43 C8.1
N$11  (via drill 0.4 pad 0.81)
  Top 0.305: R11.1 40.01,26.35 40.96,27.3 v41.59,27.3
  Bottom 0.305: v41.59,27.3 40.96,27.3 40.01,28.26 J1.4
N$12
  Top 0.305: C30.1 68.56,83.15 Y3.P$2 68.31,80.71 U2.8
N$13
  Top 0.305: C29.1 66.06,83.15 Y3.P$1 67.04,79.98 U2.9
N$14  (via drill 0.4 pad 0.81)
  Top 0.305: R19.2 13.87,6.03 12.38,6.03 11.11,7.3 11.11,17.46 8.89,19.68 8.89,28.89 10.48,30.48 55.56,30.48 v59.37,34.29 | v74.93,41.91 74.93,40.64 74.61,40.32 R14.1
  Top 0.406: R18.1 R20.1 R19.2 20.85,6.13 20.95,6.03 20.95,3.48 LIGHT_DR.2
  Bottom 0.305: v74.93,41.91 61.91,41.91 59.37,39.37 v59.37,34.29
N$15
  Bottom 0.5: D4.3 46.99,21.59 46.35,20.95 45.14,20.95 U3.16
N$16
  Bottom 0.305: D3.1 40.32,38.41 39.69,37.78 37.15,37.78 36.51,38.42 R22.1
N$18
  Bottom 0.406: D1.2 36.79,50.87 R23.2
N$19
  Top 0.254: U6.2 17.25,64 C26.1
N$20  (via drill 0.4 pad 0.81)
  Top 0.305: U2.23 60.01,62.87 60.64,63.5 60.64,64.14 v61.28,64.77
  Bottom 0.305: R49.2 R48.2 61.91,64.14 v61.28,64.77
N$21
  Top 0.305: SJR1.5 69.22,34.35 69.22,36.2 TP3.TP R31.1
N$22  (via drill 0.4 pad 0.81)
  Top 0.305: SJR1.17 62.05,31.29 v63.5,29.84 | v57.78,41.27 57.78,48.16 R17.1
  Bottom 0.305: v63.5,29.84 61.91,31.43 60.01,31.43 57.78,33.66 v57.78,41.27
N$23
  Top 0.61: R51.2 70.85,54.87 U2.33
N$24
  Top 0.61: R52.2 74.66,54.55 U2.36
N$25
  Bottom 0.813: T3.3 8.51,41.42 R38.1 8.18,41.25 LS1.-
N$26
  Bottom 0.61: R39.1 10.16,36.51 11.43,37.78 11.43,38.91 T3.1
N$27  (via drill 0.4 pad 0.81)
  Top 0.305: v31.43,39.69 30.48,39.69 29.21,40.96 29.21,44.13 27.94,45.4 v25.08,45.4
  Bottom 0.305: R41.1 30.16,40.96 v31.43,39.69 | v25.08,45.4 25.08,41.59 25.4,41.27 U$1.3
N$28
  Bottom 0.254: IC2.1 10.14,52.69 8.89,51.44 8.47,51.44 R35.2 8.26,50.8 9.53,49.53 10.58,49.53 R34.1
N$30
  Bottom 0.61: U1.1 17.09,19.74 18.1,18.73 18.1,16.85 Y2.P$2
N$31
  Bottom 0.61: Y2.P$1 15.58,19.72 U1.2
N$32
  Bottom 0.254: R36.2 IC2.3
  Bottom 0.61: R37.1 8.47,54.61 9.53,54.61 10.58,55.66 R36.2
N$33
  Bottom 0.254: C20.1 14.82,52.47 R32.2
  Bottom 0.813: R32.2 14.82,45.54 LS1.+
N$34
  Bottom 0.61: R37.2 8.26,57.71 C19.1
N$35
  Bottom 0.254: C20.2 12.28,54.22 IC2.4 R36.1
N$36
  Bottom 0.61: R39.2 7.62,36.51 4.45,39.69 4.45,55.24 5.08,55.88 5.47,55.88 C18.2 5.71,57.71 C19.2 6.13,58.13 R33.2
N$37
  Bottom 0.813: U$1.5 21.09,43.18 L1.1
N$38  (via drill 0.4 pad 0.81)
  Top 0.305: R42.2 48.36,7.62 v49.53,7.62 | v51.75,7.62 51.39,8.3 IC1.9
  Bottom 0.305: v49.53,7.62 v51.75,7.62
N$39
  Top 0.305: IC1.8 50.89,5.73 R43.1 50.7,5.51 R44.2
N$40  (via drill 0.4 pad 0.81)
  Top 0.254: R45.2 13.44,69.85 R46.1 15.34,70.7 v14.29,71.75 | U6.7 21.91,60.33 22.54,59.69 v23.5,59.69
  Bottom 0.254: v23.5,59.69 14.29,68.9 v14.29,71.75
N$41  (via drill 0.4 pad 0.81)
  Top 0.305: v66.67,55.88 65.72,56.83 65.72,58.26 U2.29
  Bottom 0.305: R50.2 66.78,61.06 65.72,60.01 65.72,56.83 v66.67,55.88
N$42
  Top 0.406: R53.2 76.83,55.88 75.93,56.78 U2.37
N$43
  Top 0.305: TP14.TP 69.85,76.58 U2.7
N$44
  Top 0.305: TP15.TP 71.12,76.58 U2.6
N$45
  Top 0.305: TP16.TP 72.39,76.58 U2.5
N$46
  Top 0.305: TP17.TP 61.91,58.26 U2.26
N$47
  Top 0.406: TP18.TP U2.17
N$48
  Top 0.406: TP19.TP U2.18
N$49
  Top 0.406: TP20.TP U2.19
N$50
  Top 0.406: TP21.TP U2.20
N$51
  Top 0.406: TP22.TP U2.21
N$52
  Top 0.406: TP23.TP U2.22
N$63
  Top 0.305: TP10.TP 60.64,76.36 U2.14
N$64
  Top 0.406: TP12.TP U2.16
N$65
  Top 0.305: TP24.TP 61.91,76.36 U2.13
N$66
  Top 0.305: U2.27 63.23,54.34 TP25.TP
N$67
  Top 0.305: TP26.TP 64.45,58.26 U2.28
N$68
  Top 0.305: U2.25 60.69,54.34 TP27.TP
NRST  (via drill 0.4 pad 0.81)
  Top 0.305: T2.3 v61.91,10.48 | v70.17,29.21 76.2,29.21 77.28,30.29 SJR1.1 77.47,34.48 77.47,37.78 76.83,38.42 R25.1 77.89,41.7 78.11,41.91 78.11,47.62 v77.79,47.94 | v74.61,74.3 74.61,76.26 U2.3
  Bottom 0.305: C16.1 69.22,21.91 | 69.22,21.91 70.17,22.86 v70.17,29.21 | v61.91,10.48 61.91,11.43 62.23,11.75 68.58,11.75 69.22,12.38 69.22,21.91 | v77.79,47.94 78.11,48.26 78.11,70.8 v74.61,74.3
PWM  (via drill 0.4 pad 0.81)
  Top 0.254: v32.07,46.99 30.8,48.26 v27.3,48.26
  Top 0.305: v76.83,51.12 R53.1
  Bottom 0.254: 9.84,60.64 14.92,55.56 15.88,55.56 16.51,54.93 16.51,49.53 17.78,48.26 v27.3,48.26
  Bottom 0.305: R13.2 R12.2 76.83,29.21 77.15,29.53 77.15,46.99 76.2,47.94 | 76.2,47.94 45.72,47.94 42.86,50.8 39.37,50.8 38.73,50.16 38.73,47.62 38.1,46.99 v32.07,46.99 | 9.84,60.64 R33.1 | 76.2,47.94 76.83,48.58 v76.83,51.12 77.15,51.44 77.15,61.59 74.61,64.14 R48.1
RTS  (via drill 0.4 pad 0.81)
  Top 0.305: v42.55,19.37 43.5,18.41 49.21,18.41 50.8,16.83 v50.8,15.88 | v54.29,15.24 53.34,15.24 52.89,14.79 IC1.24 | v63.82,8.26 63.82,6.67 62.86,5.71 T2.2
  Top 0.406: T2.2 62.97,5.14 R2.2
  Bottom 0.305: U3.14 v42.55,19.37 | v50.8,15.88 51.44,15.24 v54.29,15.24 55.56,15.24 56.2,14.61 56.2,12.38 60.33,8.26 v63.82,8.26
RXD0  (via drill 0.4 pad 0.81)
  Top 0.305: v53.98,21.59 53.87,21.49 R3.1 | SJR1.15 75.25,18.12 v75.25,20 73.34,21.91 73.34,23.18 72.71,23.81 68.9,23.81 68.9,20.95 v68.26,20.32 | U2.34 72.12,59.64 71.75,60.01 62.55,60.01 v61.28,61.28 | v40.64,53.02 39.69,52.07 39.69,42.23 40.64,41.27 43.5,41.27 43.81,40.96 v43.81,39.05
  Bottom 0.305: R7.2 49.85,17.14 50.8,18.1 50.8,21.59 | 50.8,21.59 v53.98,21.59 53.98,21.27 55.56,19.68 67.63,19.68 v68.26,20.32 | v75.25,20 76.83,20 R12.1 | 50.8,21.59 50.8,25.08 50.48,25.4 44.13,25.4 43.5,26.04 43.5,29.53 42.55,30.48 J1.3 42.55,34.92 43.81,36.2 v43.81,39.05 | v61.28,61.28 54.29,61.28 45.09,52.07 41.59,52.07 v40.64,53.02
RXD0_CP2101IN
  Top 0.305: R3.2 51.89,19.4 IC1.26
SCL  (via drill 0.4 pad 0.81)
  Top 0.254: U6.4 20.3,62.98 18.78,62.98 17.14,61.35 v17.14,34.29
  Top 0.305: 69.28,16.83 69.28,15.88 TP6.TP 69.22,12.7 68.26,11.75 65.94,11.75 R55.2 | 69.28,16.83 SJR1.12 69.22,18.15 69.22,20 v70.48,21.27 | v13.65,27.94 13.97,28.26 49.21,28.26 52.07,25.4 53.34,25.4 58.1,20.64 v58.1,17.46 | v67.31,15.88 68.33,15.88 69.28,16.83 | v66.04,40.64 66.04,50.16 69.22,53.34 69.22,56.52 68.31,57.42 U2.31
  Bottom 0.254: 72.71,28.47 72.71,33.97 | v17.14,34.29 19.37,34.29 20,33.66 20,30.8 19.37,30.16 14.92,30.16 13.65,28.89 v13.65,27.94
  Bottom 0.305: v70.48,21.27 71.12,21.91 71.12,25.72 71.44,26.04 72.71,26.04 73.56,26.89 R27.1 72.71,28.47 | U1.6 14.29,26.67 13.65,27.3 v13.65,27.94 | v58.1,17.46 58.1,15.56 66.67,15.56 v67.31,15.88 | 72.71,33.97 v66.04,40.64
SCLK  (via drill 0.4 pad 0.81)
  Top 0.305: U4.6 48.26,41.91 v53.66,36.51 | v63.5,25.4 63.5,21.91 62.87,21.27 61.3,21.27 SJR1.22
  Bottom 0.305: v53.66,36.51 53.66,33.97 58.42,29.21 59.69,29.21 v63.5,25.4
SDA  (via drill 0.4 pad 0.81)
  Top 0.254: U6.6 21.41,60.58 20.52,59.69 18.73,59.69 18.1,59.05 v18.1,32.7
  Top 0.305: v71.75,20.32 71.75,19.68 71.44,19.37 71.44,18.25 SJR1.13 71.28,16.35 TP9.TP v71.75,13.02 | v12.38,26.99 12.38,28.26 13.65,29.53 49.53,29.53 52.7,26.35 53.66,26.35 59.37,20.64 v59.37,18.73 | v71.44,40.64 71.44,50.48 v71.12,50.8 | v68.26,55.24 68.26,56.2 66.99,57.47 66.99,58.26 U2.30
  Bottom 0.254: v18.1,32.7 17.14,31.75 14.29,31.75 12.38,29.84 v12.38,26.99
  Bottom 0.305: v71.75,20.32 72.07,20.64 72.07,25.08 73.66,25.08 74.93,26.35 74.93,28.89 73.66,30.16 R29.1 73.56,38.52 v71.44,40.64 | U1.5 13.02,26.35 v12.38,26.99 | v59.37,18.73 56.83,18.73 56.83,15.24 60.64,11.11 60.64,9.53 68.9,9.53 v71.75,13.02 | v71.12,50.8 66.99,50.8 65.41,52.39 65.41,53.02 66.36,53.98 66.99,53.98 v68.26,55.24
SHIELD  (via drill 0.7 pad 0.25, 1 pad 0.1)  (3 unrouted)
  Top 0.203: J3.SHIELD6 42.17,2.42 J3.SHIELD7 | J3.SHIELD5 J3.SHIELD8 | J3.SHIELD 36.96,5.25 J3.SHIELD9 36.65,5.17 J3.SHIELD | J3.SHIELD2 41.98,5.25 J3.SHIELD10 42.29,5.17 J3.SHIELD2
  Top 0.254: J3.SHIELD2 44.62,5.25 44.77,5.4 R21.1
  Top 0.305: 44.72,5.25 R21.1 | J3.SHIELD6 36.78,2.4 J3.SHIELD5 | J3.SHIELD4 42.05,2.3 J3.SHIELD7 38.65,2.44 J3.SHIELD3
  Top 0.813: 44.77,5.4 42.23,5.4
  Bottom 0.305: J3.SHIELD5 36.74,5.08 36.65,5.17 | J3.SHIELD7 42.2,5.08 42.29,5.17 | J3.SHIELD10 42.29,5.17 | 42.29,5.17 J3.SHIELD2 | J3.SHIELD9 36.65,5.17 | 36.65,5.17 J3.SHIELD
  other vias: 37.02,5.22 41.92,5.18 42.16,2.17 36.72,2.14
  pour Bottom (isolate 0.406, no thermals): 35.56,6.03 35.56,2.22 36.2,1.59 42.23,1.59 42.86,2.22 42.86,5.71 41.59,5.71 41.59,3.49 41.27,3.17 37.78,3.17 37.47,3.49 37.47,6.03
SPI_HOLD  (via drill 0.4 pad 0.81)
  Top 0.305: SJR1.19 61.26,27.3 TP7.TP 58.74,27.3 v57.15,28.89 | v50.16,41.27 49.53,41.91 U4.7
  Bottom 0.305: v57.15,28.89 57.15,29.21 52.7,33.66 52.7,38.73 v50.16,41.27
SPI_WP  (via drill 0.4 pad 0.81)
  Top 0.305: SJR1.20 59.16,25.29 TP8.TP 58.74,25.4 v55.24,28.89 | U4.3 48.26,48.26 v45.72,45.72
  Bottom 0.305: v55.24,28.89 55.24,29.84 51.75,33.34 51.75,37.15 47.94,40.96 46.35,40.96 45.72,41.59 v45.72,45.72
SQW
  Bottom 0.61: U1.7 15.56,28.04 R16.1
TXD0  (via drill 0.4 pad 0.81)
  Top 0.305: v49.53,21.59 49.53,22.23 50.16,22.86 52.07,22.86 | 52.07,22.86 54.29,22.86 55.56,21.59 55.56,20.95 | R4.1 54.93,17.14 55.56,17.78 55.56,20.95 | 55.56,20.95 v56.2,20.95 | SJR1.16 77.28,20.2 75.25,22.23 75.25,22.54 73.03,24.77 68.26,24.77 67.31,23.81 67.31,21.27 v66.67,20.64 | 52.07,22.86 v52.07,24.13 | U2.35 73.39,60.28 72.39,61.28 62.87,61.28 v61.28,62.87 | v42.86,53.34 41.59,52.07 41.59,43.18 42.23,42.55 44.45,42.55 45.72,41.27 v45.72,39.05
  Bottom 0.305: R10.2 49.53,20.42 v49.53,21.59 | v56.2,20.95 56.2,21.27 63.18,21.27 63.82,20.64 v66.67,20.64 | v52.07,24.13 52.07,25.72 50.16,27.62 46.35,27.62 45.09,28.89 J1.2 45.09,35.56 45.72,36.2 v45.72,39.05 | v61.28,62.87 53.02,62.87 43.5,53.34 v42.86,53.34
TXD0_CP2101
  Top 0.305: R4.2 52.7,17.04 52.7,15.56 52.39,15.24 IC1.25
VBAT
  Bottom 0.61: U1.3 14.29,18.73 13.34,17.78 13.34,14.82 BT1.1
  pour Bottom (isolate 0.406, no thermals): 16.19,14.92 11.75,14.92 11.43,14.61 11.43,12.7 11.75,12.38 15.88,12.38 16.51,12.38 16.83,12.7 16.83,14.61 16.51,14.92

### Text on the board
tNames: Alarm Light v2 | Juraj Repcik | 12/2018 | X | Z | Y | * | U6 | 3V3 | GND | GND | IC1 | +5V
bNames: * | U4 | * | U1 | U3
DrillLegend: LAYER-STACK
DrillLegend_01-16: 01-16
DrillLegend_01-20: 01-20

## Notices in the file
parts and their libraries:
SparkFun-LED: Licensing: Creative Commons ShareAlike 4.0 International - https://creativecommons.org/licenses/by-sa/4.0
